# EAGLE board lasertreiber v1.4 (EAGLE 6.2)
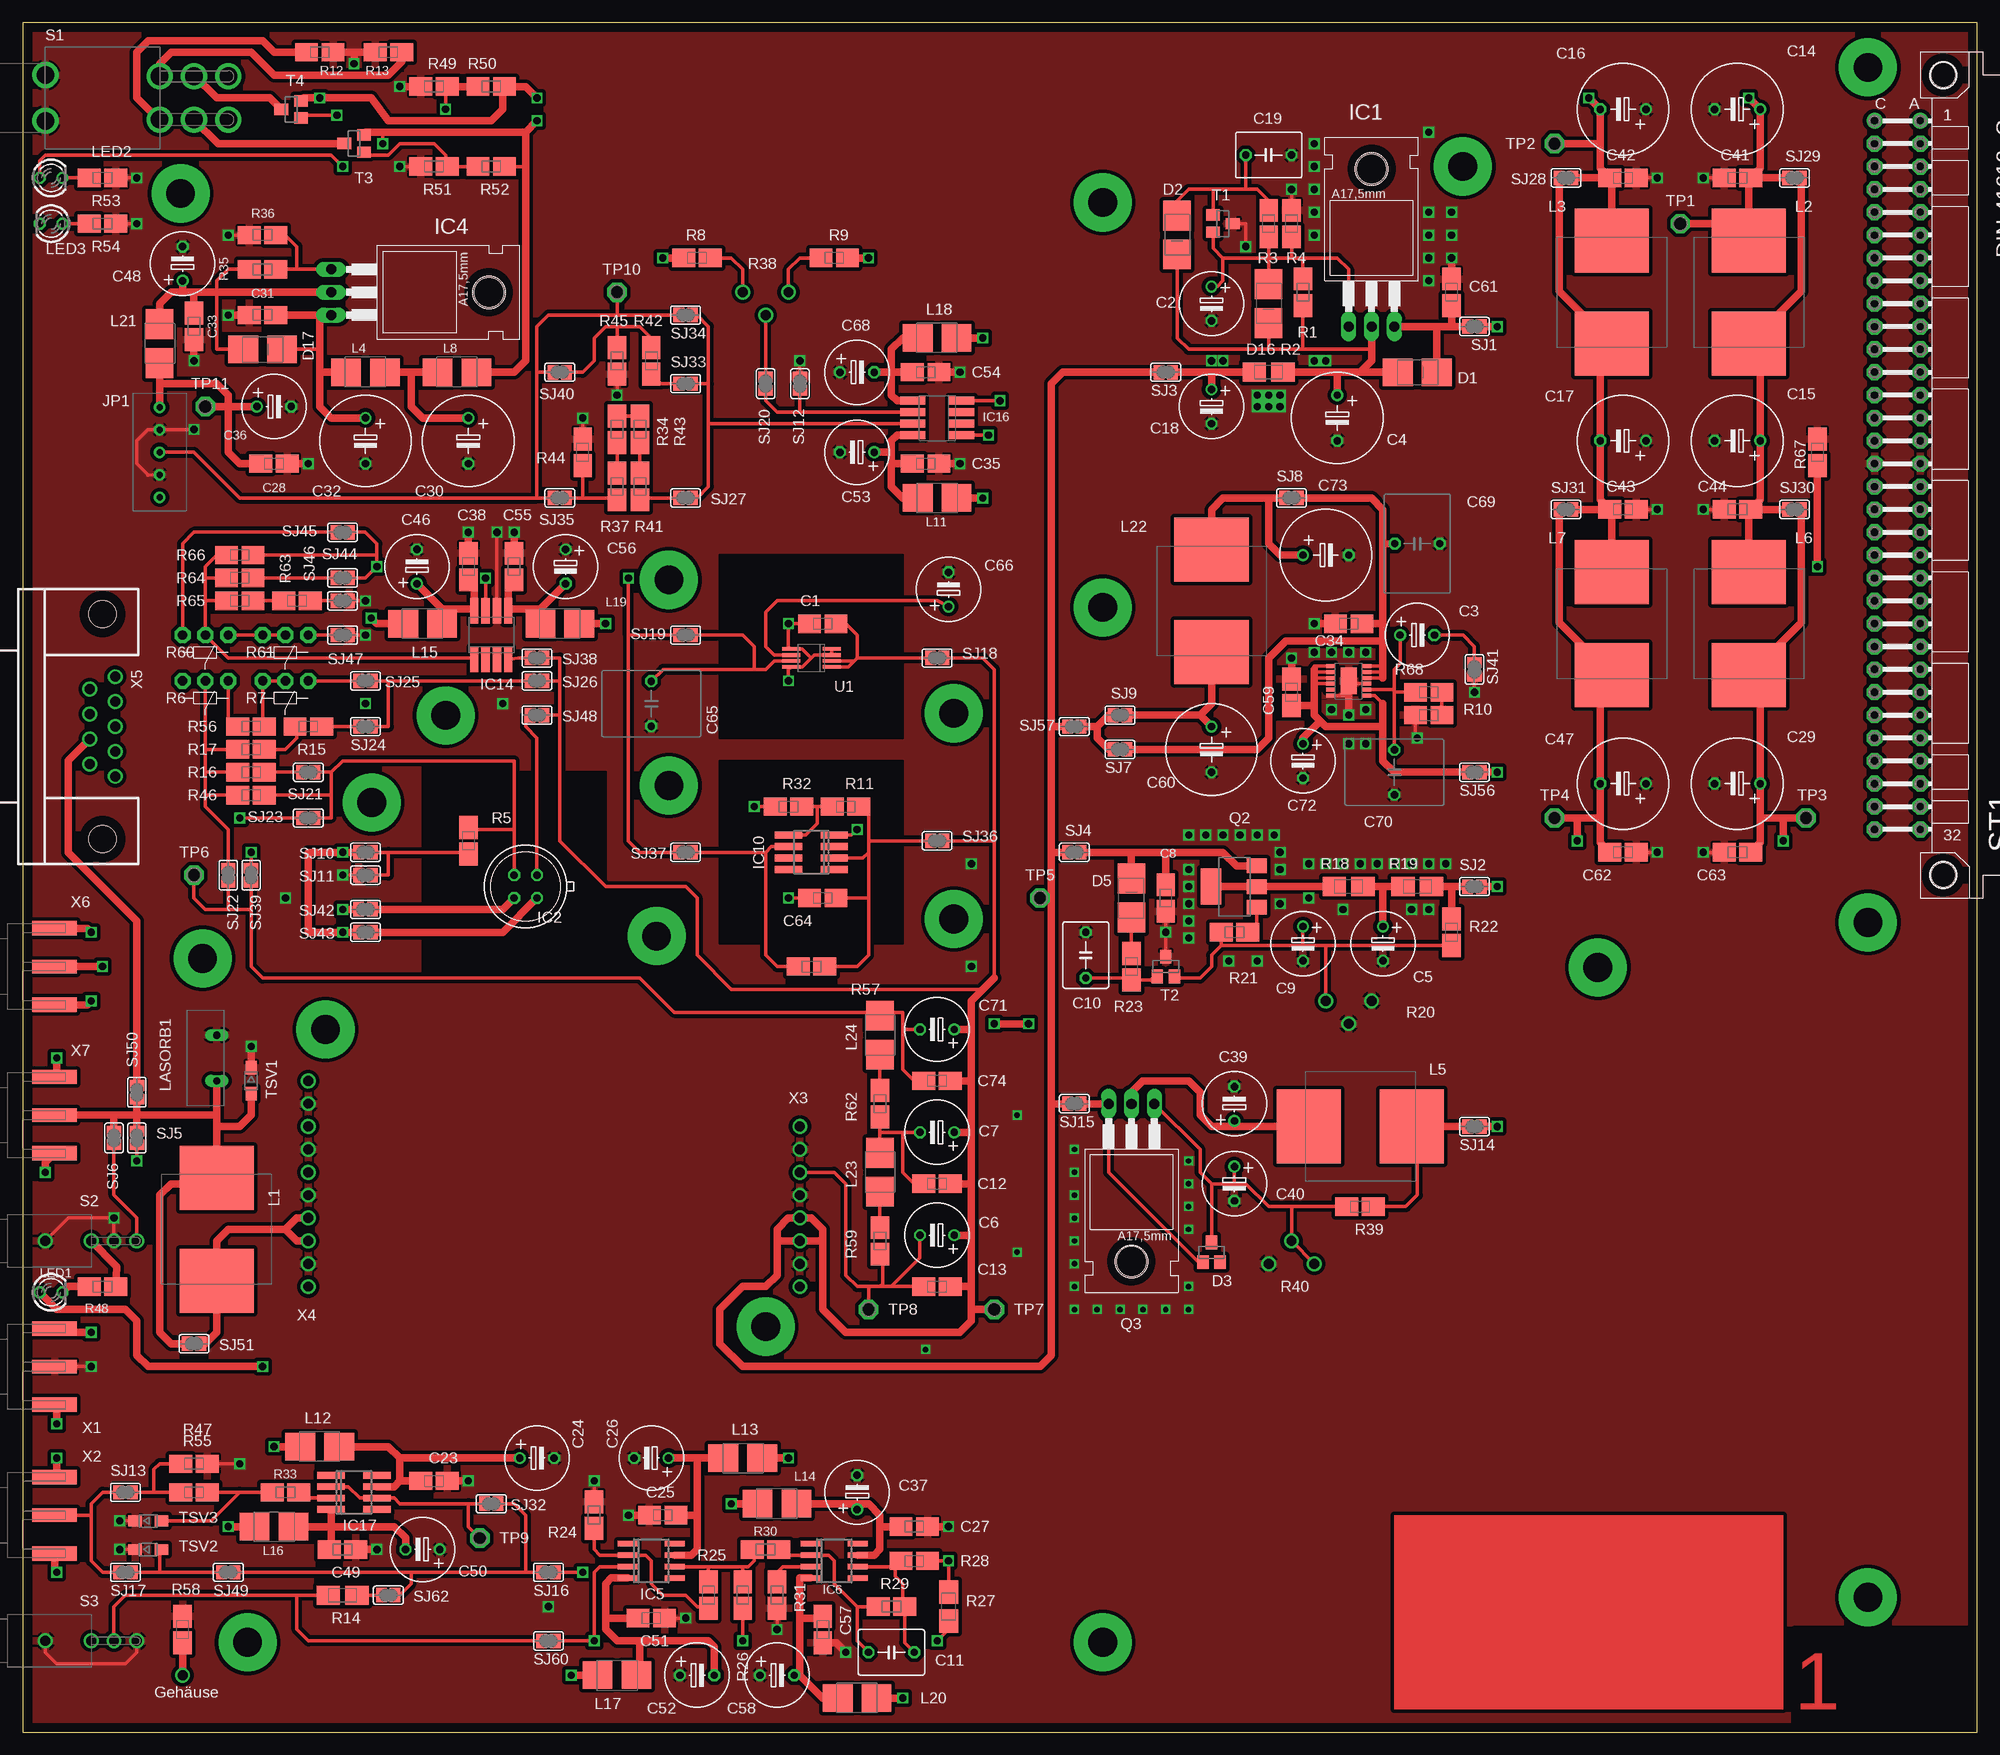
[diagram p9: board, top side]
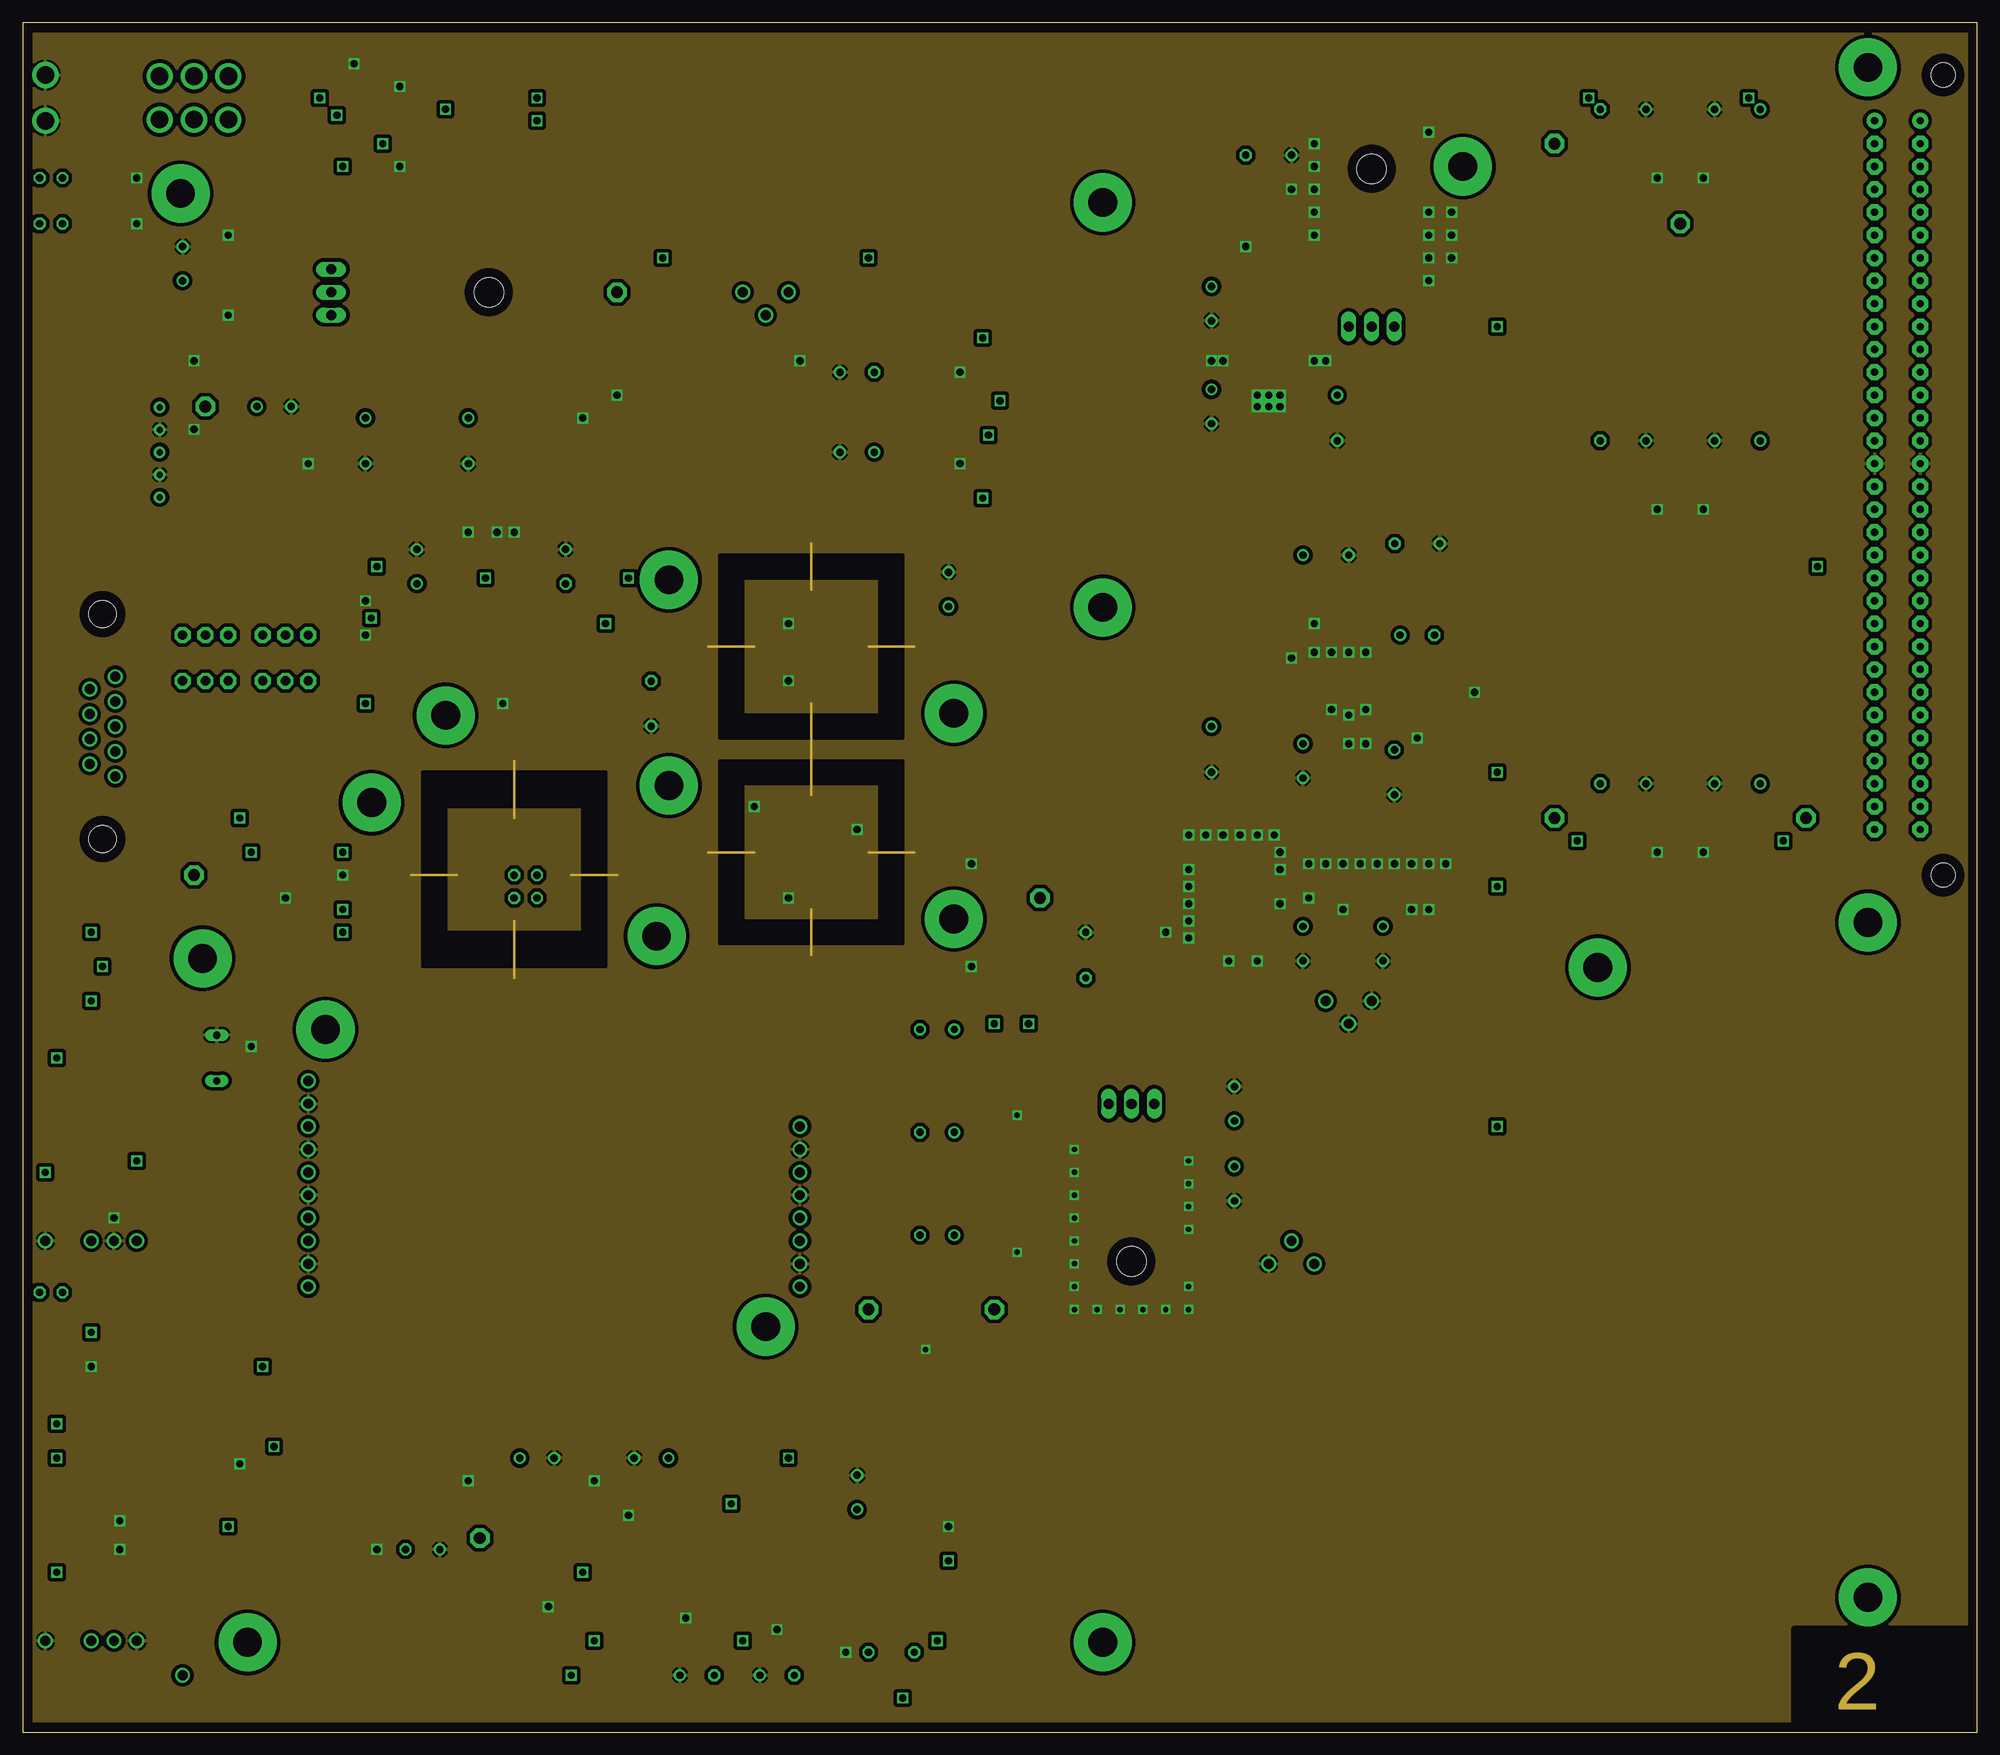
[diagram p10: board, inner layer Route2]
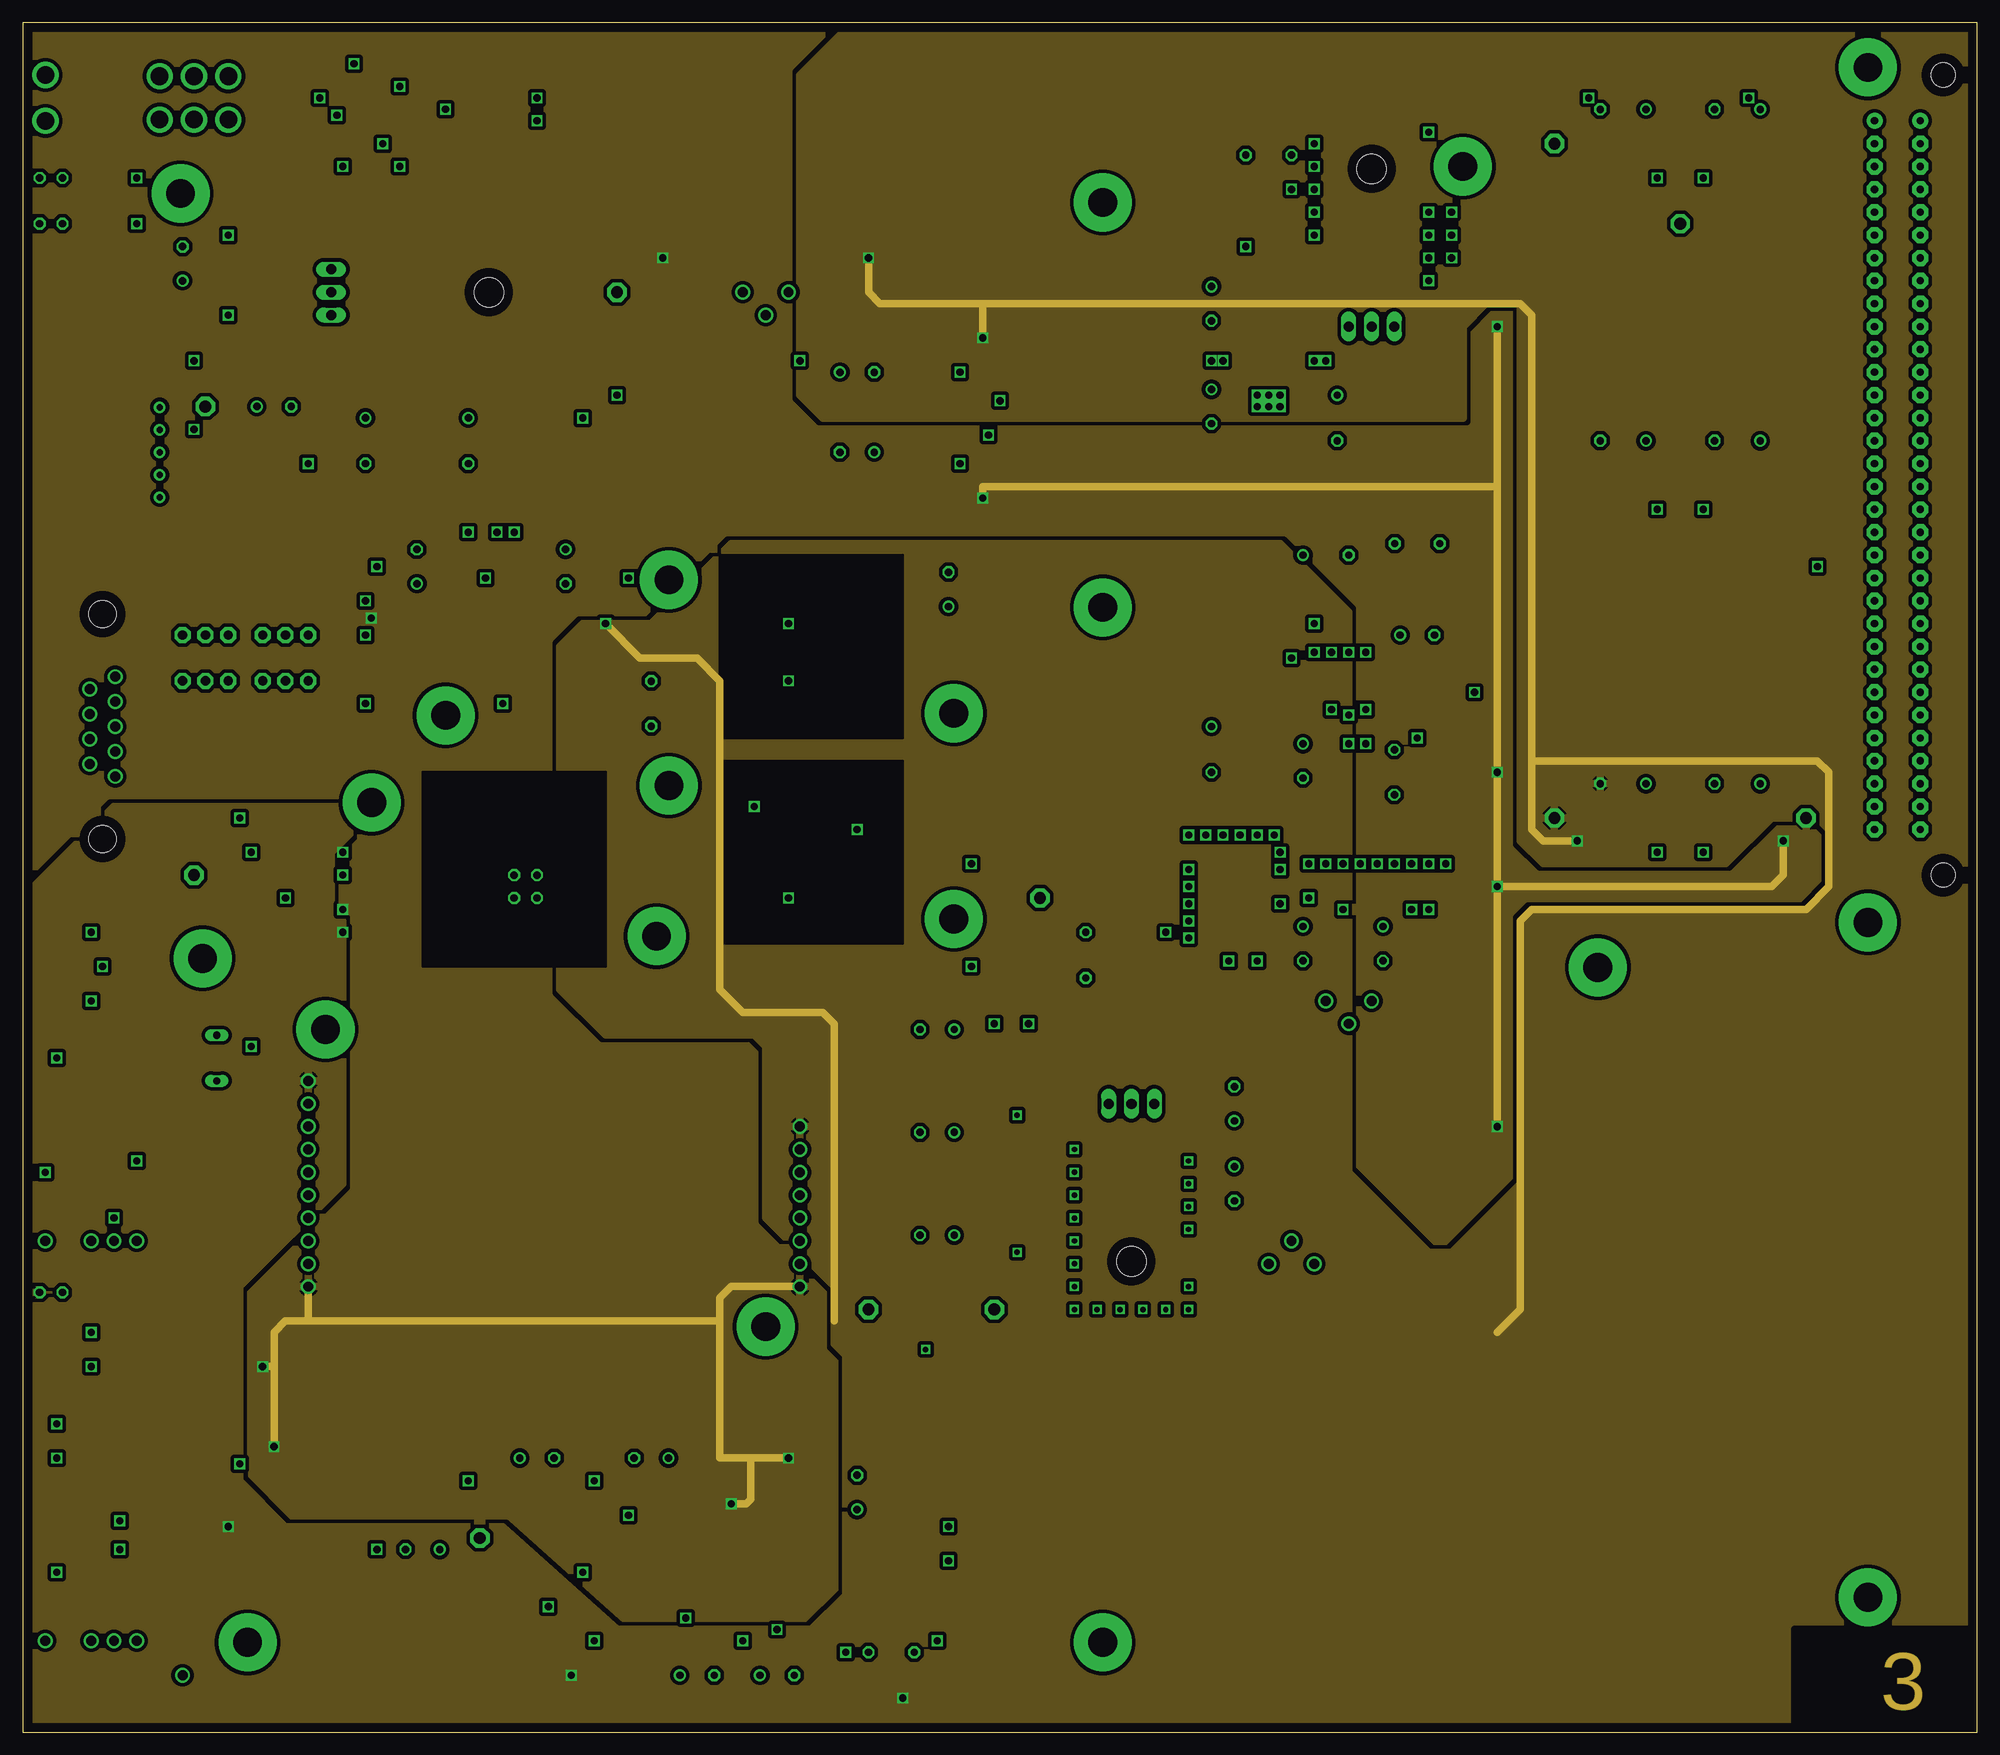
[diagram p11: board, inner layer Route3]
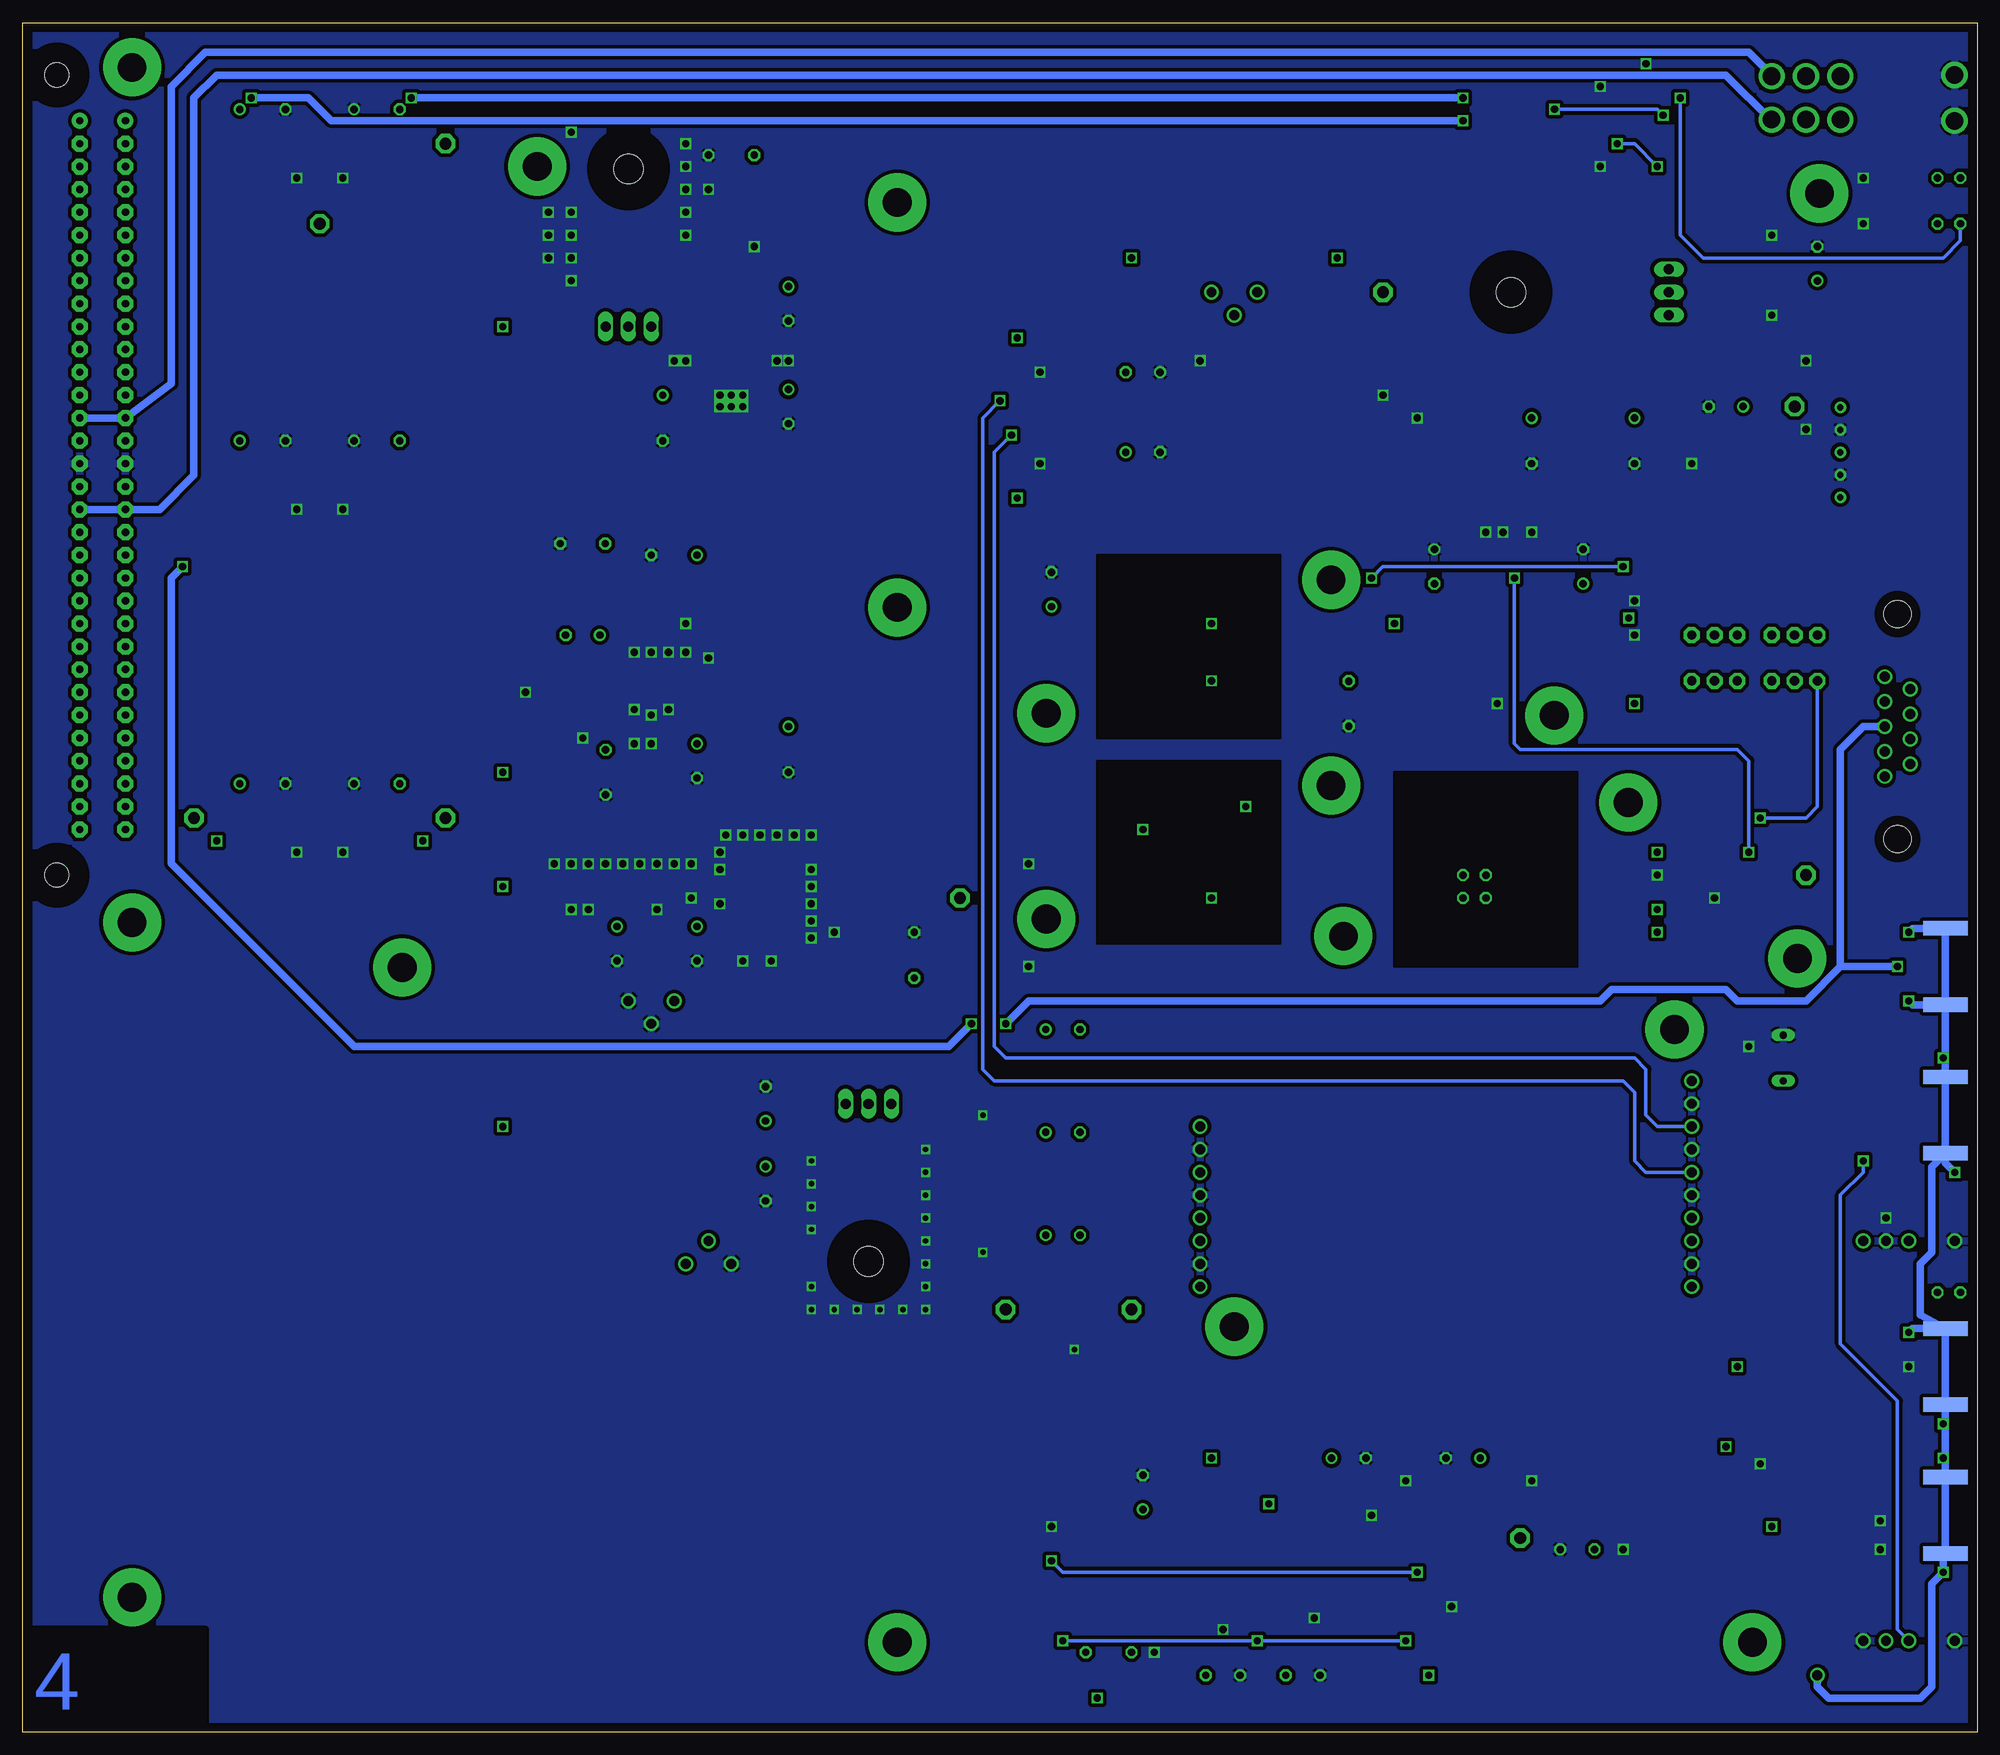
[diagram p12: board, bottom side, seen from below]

Size 217.17 x 189.99 mm. Coordinates in mm from the lower left corner, seen from the top.
Outline: 0,0 217.17,0 217.17,189.99 0,189.99 0,0
Copper layers (1+2*3+16): Top 0.018mm / dielectric 0.14mm / Route2 0.035mm / dielectric 1.2mm / Route3 0.035mm / dielectric 0.14mm / Bottom 0.018mm
Design rules: minimum track width 10mil, minimum drill 23mil, track to track 8mil, track to pad 8mil, pad to pad 8mil, via to via 8mil, smd to smd 8mil, copper to edge 40mil, drill to drill 8mil, minimum pad ring 10mil, minimum via ring 8mil, stop-mask expansion 4mil, vias tented up to drill 0mil, thermal gap 10mil

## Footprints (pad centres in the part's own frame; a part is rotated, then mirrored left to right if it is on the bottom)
LOCH-M3 = drill 3.2 pad 6.452: 1 0,0
BOX-15X15MM = drill 3.2 pad 6.452: 1 -15.824,7.417; 2 15.824,-7.417
C0805 = smd 2.54 x 2.032: 1 -1.473,0; 2 1.473,0
TT5D7 = drill 0.813: + -1.905,0 | drill 0.813 octagon: - 1.905,0
TT5D10 = drill 0.813: + -2.54,0 | drill 0.813 octagon: - 2.54,0
C050-050X075 = drill 0.813 octagon: 1 -2.54,0; 2 2.54,0
MKS2 = drill 0.813 octagon: 1 -2.5,0; 2 2.5,0
DIODE = smd 3.302 x 3.048: ANODE -2.159,0; KATHODE 2.159,0
SOT23 = smd 1.27 x 1.524: 1 -0.95,-1.1; 2 0.95,-1.1; 3 0,1.1
GEHAEUSEMASSE = drill 1.1: P$2 0,0
TO220 = drill 1.118 long: 1 -2.54,-6.35; 2 0,-6.35; 3 2.54,-6.35 | hole 3.302: 0,11.176
TO39/4 = drill 0.813 octagon: 1 -1.27,-1.27; 2 1.27,-1.27; 3 1.27,1.27; 4 -1.27,1.27
MSE = smd 0.445 x 1.016: 1 -1.626,-2; 2 -0.975,-2; 3 -0.325,-2; 4 0.325,-2; 5 0.975,-2; 6 1.626,-2; 7 1.626,2; 8 0.975,2; 9 0.325,2; 10 -0.325,2; 11 -0.975,2; 12 -1.626,2 | smd 2.9 x 1.75: 13 0,0
SO08 = smd 0.6 x 2.2: 1 -1.905,-2.6; 2 -0.635,-2.6; 3 0.635,-2.6; 4 1.905,-2.6; 5 1.905,2.6; 6 0.635,2.6; 7 -0.635,2.6; 8 -1.905,2.6
SOIC8 = smd 0.762 x 3.048: 1 -1.905,-2.54; 2 -0.635,-2.54; 3 0.635,-2.54; 4 1.905,-2.54; 5 1.905,2.54; 6 0.635,2.54; 7 -0.635,2.54; 8 -1.905,2.54
R-8 = smd 0.9 x 2.8: 1 -1.905,-2.7; 2 -0.635,-2.7; 3 0.635,-2.7; 4 1.905,-2.7; 5 1.905,2.7; 6 0.635,2.7; 7 -0.635,2.7; 8 -1.905,2.7
IL-G5 = drill 0.7 pad 1.27: P$1 0,5; P$2 0,2.5; P$3 0,0; P$4 0,-2.5; P$5 0,-5
L-GROSS = smd 7.112 x 8.23: P$1 -5.715,0; P$2 5.715,0
L-KLEIN = smd 3.302 x 3.048: 1 -2.159,0; 2 2.159,0
LASORB = drill 0.8 long: LDA 2.54,0; LDK -2.54,0
LED3MM = drill 0.813 octagon: A -1.27,0; K 1.27,0
SOT223 = smd 1.6 x 2.2: 1 -2.3,-2.5; 2 0,-2.5; 3 2.3,-2.5 | smd 4 x 2.3: 4 0,2.6
R0805 = smd 2.54 x 2.032: 1 -1.473,0; 2 1.473,0
R1206 = smd 2.6 x 2.1: 1 -1.6,0; 2 1.6,0
PT-10 = drill 1.016 pad 1.778 octagon: 1 -2.54,1.27; 2 2.54,1.27; 3 0,1.27
64Y-POTI = drill 1.1: 1 2.54,-1.27; 2 0,1.27; 3 -2.54,-1.27
1MD1T2B4M7QE = drill 1.95: 1 -2.413,0; 2 -2.413,3.81; 3 -2.413,7.62; 4 2.413,0; 5 2.413,3.81; 6 2.413,7.62; 7 -2.54,-12.7; 8 2.54,-12.7
2AS1T2A1M7RE = drill 1.1: 1 0,0; 2 0,2.54; 3 0,5.08; 4 0,-5.08
SJ = smd 1.168 x 1.6: 1 -0.762,0; 2 0.762,0
A.KO-09_MAC64L = drill 0.8 pad 1.778: A1 -1.27,39.37; C1 -6.35,39.37 | drill 0.8 pad 1.778 octagon: A2 -1.27,36.83; A3 -1.27,34.29; A4 -1.27,31.75; A5 -1.27,29.21; A6 -1.27,26.67; A7 -1.27,24.13; A8 -1.27,21.59; A9 -1.27,19.05; A10 -1.27,16.51; A11 -1.27,13.97; A12 -1.27,11.43; A13 -1.27,8.89; A14 -1.27,6.35; A15 -1.27,3.81; A16 -1.27,1.27; A17 -1.27,-1.27; A18 -1.27,-3.81; A19 -1.27,-6.35; A20 -1.27,-8.89; A21 -1.27,-11.43; A22 -1.27,-13.97; A23 -1.27,-16.51; A24 -1.27,-19.05; A25 -1.27,-21.59; A26 -1.27,-24.13; A27 -1.27,-26.67; A28 -1.27,-29.21; A29 -1.27,-31.75; A30 -1.27,-34.29; A31 -1.27,-36.83; A32 -1.27,-39.37; C2 -6.35,36.83; C3 -6.35,34.29; C4 -6.35,31.75; C5 -6.35,29.21; C6 -6.35,26.67; C7 -6.35,24.13; C8 -6.35,21.59; C9 -6.35,19.05; C10 -6.35,16.51; C11 -6.35,13.97; C12 -6.35,11.43; C13 -6.35,8.89; C14 -6.35,6.35; C15 -6.35,3.81; C16 -6.35,1.27; C17 -6.35,-1.27; C18 -6.35,-3.81; C19 -6.35,-6.35; C20 -6.35,-8.89; C21 -6.35,-11.43; C22 -6.35,-13.97; C23 -6.35,-16.51; C24 -6.35,-19.05; C25 -6.35,-21.59; C26 -6.35,-24.13; C27 -6.35,-26.67; C28 -6.35,-29.21; C29 -6.35,-31.75; C30 -6.35,-34.29; C31 -6.35,-36.83; C32 -6.35,-39.37 | hole 2.7: 1.27,44.45; 1.27,-44.45
P1-13 = drill 1.321 pad 2.159 octagon: TP 0,0
SOD323-W = smd 1.5 x 1.2: A 1.45,0; C -1.45,0
MS8 = smd 0.4 x 2: 1 -1,-2.25; 2 -0.325,-2.25; 3 0.325,-2.25; 4 1,-2.25; 5 1,2.25; 6 0.325,2.25; 7 -0.325,2.25; 8 -1,2.25
SMA20_HRZ = smd 1.6 x 4.902 bottom: GND@1 -4.242,3.556; GND@4 4.242,3.556 | smd 1.6 x 4.902: GND@2 -4.242,3.556; GND@3 4.242,3.556 | smd 1.499 x 4.902: SIGNAL 0,3.556
PINHEADER-8 = drill 1.1: 1 -8.89,0; 2 -6.35,0; 3 -3.81,0; 4 -1.27,0; 5 1.27,0; 6 3.81,0; 7 6.35,0; 8 8.89,0
PINHEADER-10 = drill 1.1: 1 -11.43,0; 2 -8.89,0; 3 -6.35,0; 4 -3.81,0; 5 -1.27,0; 6 1.27,0; 7 3.81,0; 8 6.35,0; 9 8.89,0; 10 11.43,0
H3M09RA = drill 1.092: 1 -5.537,1.422; 2 -2.769,1.422; 3 0,1.422; 4 2.769,1.422; 5 5.537,1.422; 6 -4.153,-1.422; 7 -1.384,-1.422; 8 1.384,-1.422; 9 4.153,-1.422 | hole 3.048: -12.497,0; 12.497,0

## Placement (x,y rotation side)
BOLZEN1  BOLZEN-M3  [LOCH-M3]  17.56,171 0 top
BOLZEN2  BOLZEN-M3  [LOCH-M3]  25,10 0 top
BOLZEN3  BOLZEN-M3  [LOCH-M3]  47,113 0 top
BOLZEN4  BOLZEN-M3  [LOCH-M3]  120,10 0 top
BOLZEN5  BOLZEN-M3  [LOCH-M3]  120,125 0 top
BOLZEN6  BOLZEN-M3  [LOCH-M3]  205,15 0 top
BOLZEN7  BOLZEN-M3  [LOCH-M3]  120,170 0 top
BOLZEN8  BOLZEN-M3  [LOCH-M3]  205,90 0 top
BOLZEN9  BOLZEN-M3  [LOCH-M3]  160,174 270 top
BOLZEN10  BOLZEN-M3  [LOCH-M3]  20,86 0 top
BOLZEN11  BOLZEN-M3  [LOCH-M3]  175,85 0 top
BOLZEN12  BOLZEN-M3  [LOCH-M3]  205,185 0 top
BOLZEN13  BOLZEN-M3  [LOCH-M3]  82.55,45.09 90 top
BOLZEN14  BOLZEN-M3  [LOCH-M3]  33.66,78.11 0 top
BOX1  BOX15X15MM  [BOX-15X15MM]  54.61,95.89 0 top
BOX2  BOX15X15MM  [BOX-15X15MM]  87.63,120.65 0 top
BOX3  BOX15X15MM  [BOX-15X15MM]  87.63,97.79 0 top
C1  100n  [C0805]  88.9,123.19 180 top
C2  100u  [TT5D7]  132.08,158.75 270 top
C3  100u  [TT5D7]  154.94,121.92 0 top
C4  1000u  [TT5D10]  146.05,146.05 270 top
C5  100u  [TT5D7]  151.13,87.63 270 top
C6  100u  [TT5D7]  101.6,55.24 180 top
C7  100u  [TT5D7]  101.6,66.67 180 top
C8  100n  [C0805]  127,92.71 90 top
C9  100u  [TT5D7]  142.24,87.63 270 top
C10  1u  [C050-050X075]  118.11,86.36 270 top
C11  1u  [C050-050X075]  96.52,8.89 0 top
C12  100n  [C0805]  101.6,60.96 0 top
C13  100n  [C0805]  101.6,49.53 0 top
C14  1000u  [TT5D10]  190.5,180.34 180 top
C15  1000u  [TT5D10]  190.5,143.51 180 top
C16  1000u  [TT5D10]  177.8,180.34 180 top
C17  1000u  [TT5D10]  177.8,143.51 180 top
C18  100u  [TT5D7]  132.08,147.32 270 top
C19  1u  [C050-050X075]  138.43,175.26 180 top
C23  100n  [C0805]  45.72,27.94 0 top
C24  100u  [TT5D7]  57.15,30.48 0 top
C25  100n  [C0805]  71.12,24.13 180 top
C26  100u  [TT5D7]  69.85,30.48 180 top
C27  100n  [C0805]  99.06,22.86 0 top
C28  100n  [C0805]  27.94,140.97 0 top
C29  1000u  [TT5D10]  190.5,105.41 180 top
C30  1000u  [TT5D10]  49.53,143.51 270 top
C31  100n  [C0805]  26.67,157.48 180 top
C32  1000u  [TT5D10]  38.1,143.51 270 top
C33  100n  [C0805]  19.05,156.21 270 top
C34  100n  [C0805]  147.32,123.19 0 top
C35  100n  [C0805]  100.33,140.97 0 top
C36  100u  [TT5D7]  27.94,147.32 0 top
C37  100u  [TT5D7]  92.71,26.67 90 top
C38  100n  [C0805]  49.53,129.54 90 top
C39  100u  [TT5D7]  134.62,69.85 90 top
C40  100u  [TT5D7]  134.62,60.96 270 top
C41  100n  [C0805]  190.5,172.72 180 top
C42  100n  [C0805]  177.8,172.72 180 top
C43  100n  [C0805]  177.8,135.89 180 top
C44  100n  [C0805]  190.5,135.89 180 top
C46  100u  [TT5D7]  43.81,129.54 90 top
C47  1000u  [TT5D10]  177.8,105.41 180 top
C48  100u  [TT5D7]  17.78,163.19 90 top
C49  100n  [C0805]  35.56,20.32 0 top
C50  100u  [TT5D7]  44.45,20.32 180 top
C51  100n  [C0805]  69.85,12.7 0 top
C52  100u  [TT5D7]  74.93,6.35 0 top
C53  100u  [TT5D7]  92.71,142.24 180 top
C54  100n  [C0805]  100.33,151.13 0 top
C55  100n  [C0805]  54.61,129.54 90 top
C56  100u  [TT5D7]  60.33,129.54 270 top
C57  100n  [C0805]  88.9,11.43 270 top
C58  100u  [TT5D7]  83.82,6.35 0 top
C59  100n  [C0805]  140.97,115.57 270 top
C60  1000u  [TT5D10]  132.08,109.22 270 top
C61  100n  [C0805]  158.75,160.02 270 top
C62  100n  [C0805]  177.8,97.79 180 top
C63  100n  [C0805]  190.5,97.79 180 top
C64  100n  [C0805]  88.9,92.71 180 top
C65  10u  [MKS2]  69.85,114.3 270 top
C66  100u  [TT5D7]  102.87,127 90 top
C68  100u  [TT5D7]  92.71,151.13 0 top
C69  10u  [MKS2]  154.94,132.08 180 top
C70  10u  [MKS2]  152.4,106.68 90 top
C71  100u  [TT5D7]  101.6,78.11 180 top
C72  100u  [TT5D7]  142.24,107.95 270 top
C73  1000u  [TT5D10]  144.78,130.81 0 top
C74  100n  [C0805]  101.6,72.39 0 top
D1  DIODEM6  [DIODE]  154.94,151.13 0 top
D2  DIODEM6  [DIODE]  128.27,166.37 270 top
D3  BZX84-A12  [SOT23]  132.08,53.34 0 top
D5  DIODEM6  [DIODE]  123.19,92.71 90 top
D16  DIODEM6  [DIODE]  138.43,158.75 270 top
D17  DIODEM6  [DIODE]  26.67,153.67 0 top
GEHAEUSE1  GEHAEUSEMASSE  [GEHAEUSEMASSE]  17.78,6.35 0 top
IC1  LM317KCS  [TO220]  149.86,162.56 0 top
IC2  LM399H  [TO39/4]  55.88,93.98 180 top
IC3  LT3045  [MSE]  147.32,116.84 270 top
IC4  LM317KCS  [TO220]  40.64,160.02 270 top
IC5  OP27D  [SO08]  69.85,19.05 270 top
IC6  OP27D  [SO08]  90.17,19.05 270 top
IC10  LT1236S-10  [SOIC8]  87.63,97.79 90 top
IC14  AD8429  [R-8]  52.07,121.92 0 top
IC16  AD8429  [R-8]  101.6,146.05 90 top
IC17  LT1028  [SOIC8]  36.83,26.67 270 top
JP1  IL-G5  [IL-G5]  15.24,142.24 180 top
L1  100u  [L-GROSS]  21.59,55.88 90 top
L2  100u  [L-GROSS]  191.77,160.02 270 top
L3  100u  [L-GROSS]  176.53,160.02 270 top
L4  100u  [L-KLEIN]  38.1,151.13 180 top
L5  100u  [L-GROSS]  148.59,67.31 180 top
L6  100u  [L-GROSS]  191.77,123.19 270 top
L7  100u  [L-GROSS]  176.53,123.19 270 top
L8  100u  [L-KLEIN]  48.26,151.13 180 top
L11  100u  [L-KLEIN]  101.6,137.16 0 top
L12  100u  [L-KLEIN]  33.02,31.75 180 top
L13  100u  [L-KLEIN]  80.01,30.48 0 top
L14  100u  [L-KLEIN]  83.82,25.4 180 top
L15  100u  [L-KLEIN]  44.45,123.19 180 top
L16  100u  [L-KLEIN]  27.94,22.86 0 top
L17  100u  [L-KLEIN]  66.04,6.35 0 top
L18  100u  [L-KLEIN]  101.6,154.94 180 top
L19  100u  [L-KLEIN]  59.69,123.19 180 top
L20  100u  [L-KLEIN]  92.71,3.81 180 top
L21  100u  [L-KLEIN]  15.24,154.31 270 top
L22  100u  [L-GROSS]  132.08,125.73 270 top
L23  100u  [L-KLEIN]  95.25,62.23 270 top
L24  100u  [L-KLEIN]  95.25,77.47 270 top
LASORB1  LASORB  [LASORB]  21.59,74.93 270 top
LED1  GRUEN  [LED3MM]  3.17,48.9 0 top
LED2  GRUEN  [LED3MM]  3.17,172.72 0 top
LED3  GRUEN  [LED3MM]  3.17,167.64 180 top
Q2  BCP56  [SOT223]  134.62,93.98 90 top
Q3  IRF512  [TO220]  123.19,63.5 180 top
R1  330R  [R0805]  142.24,160.02 270 top
R2  4R7  [R1206]  138.43,151.13 0 top
R3  51k  [R0805]  138.43,167.64 90 top
R4  3k3  [R0805]  140.97,167.64 270 top
R5  7.5k  [R0805]  49.53,99.06 90 top
R6  10k  [PT-10]  20.32,115.57 0 top
R7  100k  [PT-10]  29.21,115.57 0 top
R8  10k  [R0805]  74.93,163.83 180 top
R9  10k  [R0805]  90.17,163.83 180 top
R10  20k  [R0805]  156.21,113.03 0 top
R11  4k7  [R0805]  91.44,102.87 180 top
R12  10R  [R0805]  33.02,186.69 0 top
R13  10R  [R0805]  40.64,186.69 180 top
R14  1k  [R1206]  35.56,15.24 0 top
R15  [R0805]  31.75,111.76 0 top
R16  [R0805]  25.4,106.68 180 top
R17  [R0805]  25.4,109.22 0 top
R18  4R7  [R1206]  147.32,93.98 0 top
R19  4R7  [R1206]  154.94,93.98 0 top
R20  10k  [64Y-POTI]  147.32,80.01 180 top
R21  10R  [R0805]  134.62,88.9 180 top
R22  10k  [R0805]  158.75,88.9 90 top
R23  51k  [R0805]  123.19,85.09 270 top
R24  1k  [R0805]  63.5,24.13 90 top
R25  1k  [R0805]  76.2,15.24 270 top
R26  1k  [R0805]  80.01,15.24 270 top
R27  1k  [R1206]  102.87,13.97 90 top
R28  2k  [R0805]  99.06,19.05 180 top
R29  1k  [R0805]  96.52,13.97 180 top
R30  1k  [R0805]  82.55,20.32 180 top
R31  1k  [R0805]  83.82,15.24 270 top
R32  4k7  [R0805]  85.09,102.87 180 top
R33  250R  [R0805]  29.21,26.67 0 top
R34  10k  [R0805]  66.04,144.78 90 top
R35  330R  [R0805]  26.67,162.56 180 top
R36  1k  [R0805]  26.67,166.37 0 top
R37  10k  [R0805]  66.04,138.43 90 top
R38  1k  [64Y-POTI]  82.55,158.75 180 top
R39  1k  [R0805]  148.59,58.42 0 top
R40  100k  [64Y-POTI]  140.97,53.34 0 top
R41  10k  [R0805]  68.58,138.43 270 top
R42  10k  [R0805]  69.85,152.4 270 top
R43  10k  [R0805]  68.58,144.78 270 top
R44  10k  [R0805]  62.23,142.24 270 top
R45  10k  [R0805]  66.04,152.4 90 top
R46  1M  [R0805]  25.4,104.14 180 top
R47  49R9  [R0805]  19.05,29.84 180 top
R48  10k  [R0805]  8.89,49.53 0 top
R49  100k  [R0805]  45.72,182.88 180 top
R50  100k  [R0805]  52.07,182.88 180 top
R51  100k  [R0805]  45.72,173.99 0 top
R52  100k  [R0805]  52.07,173.99 0 top
R53  10k  [R0805]  8.89,172.72 0 top
R54  10k  [R0805]  8.89,167.64 0 top
R55  250R  [R0805]  19.05,26.67 0 top
R56  [R0805]  25.4,111.76 0 top
R57  1M  [R0805]  87.63,85.09 180 top
R58  0R  [R0805]  17.78,11.43 90 top
R59  1k  [R0805]  95.25,54.61 270 top
R60  10k  [PT-10]  20.32,120.65 0 top
R61  100k  [PT-10]  29.21,120.65 0 top
R62  1k  [R0805]  95.25,69.85 270 top
R63  [R0805]  30.48,125.73 0 top
R64  [R0805]  24.13,128.27 180 top
R65  [R0805]  24.13,125.73 0 top
R66  1M  [R0805]  24.13,130.81 180 top
R67  0R  [R0805]  199.39,142.24 90 top
R68  100k  [R0805]  156.21,115.57 180 top
S1  1MD1T2B4M7QE  [1MD1T2B4M7QE]  15.24,181.61 270 top
S2  2AS1T2A1M7RE  [2AS1T2A1M7RE]  7.62,54.61 270 top
S3  2AS1T2A1M7RE  [2AS1T2A1M7RE]  7.62,10.16 270 top
SJ1  [SJ]  161.29,156.21 180 top
SJ2  [SJ]  161.29,93.98 180 top
SJ3  [SJ]  127,151.13 180 top
SJ4  [SJ]  116.84,97.79 180 top
SJ5  [SJ]  12.7,66.04 90 top
SJ6  [SJ]  10.16,66.04 270 top
SJ7  [SJ]  121.92,109.22 180 top
SJ8  [SJ]  140.97,137.16 180 top
SJ9  [SJ]  121.92,113.03 180 top
SJ10  [SJ]  38.1,97.79 180 top
SJ11  [SJ]  38.1,95.25 180 top
SJ12  [SJ]  86.36,149.86 90 top
SJ13  [SJ]  11.43,26.67 0 top
SJ14  [SJ]  161.29,67.31 180 top
SJ15  [SJ]  116.84,69.85 180 top
SJ16  [SJ]  58.42,17.78 0 top
SJ17  [SJ]  11.43,17.78 0 top
SJ18  [SJ]  101.6,119.38 0 top
SJ19  [SJ]  73.66,121.92 180 top
SJ20  [SJ]  82.55,149.86 90 top
SJ21  [SJ]  31.75,106.68 180 top
SJ22  [SJ]  22.86,95.25 270 top
SJ23  [SJ]  31.75,101.6 180 top
SJ24  [SJ]  38.1,111.76 0 top
SJ25  [SJ]  38.1,116.84 0 top
SJ26  [SJ]  57.15,116.84 0 top
SJ27  [SJ]  73.66,137.16 180 top
SJ28  [SJ]  171.45,172.72 180 top
SJ29  [SJ]  196.85,172.72 0 top
SJ30  [SJ]  196.85,135.89 0 top
SJ31  [SJ]  171.45,135.89 180 top
SJ32  [SJ]  52.07,25.4 0 top
SJ33  [SJ]  73.66,149.86 180 top
SJ34  [SJ]  73.66,157.48 180 top
SJ35  [SJ]  59.69,137.16 180 top
SJ36  [SJ]  101.6,99.06 0 top
SJ37  [SJ]  73.66,97.79 180 top
SJ38  [SJ]  57.15,119.38 180 top
SJ39  [SJ]  25.4,95.25 270 top
SJ40  [SJ]  59.69,151.13 180 top
SJ41  [SJ]  161.29,118.11 90 top
SJ42  [SJ]  38.1,91.44 180 top
SJ43  [SJ]  38.1,88.9 0 top
SJ44  [SJ]  35.56,128.27 180 top
SJ45  [SJ]  35.56,133.35 180 top
SJ46  [SJ]  35.56,125.73 0 top
SJ47  [SJ]  35.56,121.92 0 top
SJ48  [SJ]  57.15,113.03 0 top
SJ49  [SJ]  22.86,17.78 0 top
SJ50  [SJ]  12.7,71.12 90 top
SJ51  [SJ]  19.05,43.18 0 top
SJ56  [SJ]  161.29,106.68 180 top
SJ57  [SJ]  116.84,111.76 180 top
SJ60  [SJ]  58.42,10.16 180 top
SJ62  [SJ]  40.64,15.24 180 top
ST1  [A.KO-09_MAC64L]  212.09,139.7 0 top
T1  BC857C  [SOT23]  133.35,167.64 270 top
T2  BC857C  [SOT23]  127,85.09 0 top
T3  IRLML9301  [SOT23]  36.83,176.53 90 top
T4  IRLML0060  [SOT23]  29.84,180.34 90 top
TP1  PTR1PAD1-13  [P1-13]  184.15,167.64 0 top
TP2  PTR1PAD1-13  [P1-13]  170.18,176.53 0 top
TP3  PTR1PAD1-13  [P1-13]  198.12,101.6 0 top
TP4  PTR1PAD1-13  [P1-13]  170.18,101.6 0 top
TP5  PTR1PAD1-13  [P1-13]  113.03,92.71 0 top
TP6  PTR1PAD1-13  [P1-13]  19.05,95.25 270 top
TP7  PTR1PAD1-13  [P1-13]  107.95,46.99 0 top
TP8  PTR1PAD1-13  [P1-13]  93.98,46.99 0 top
TP9  PTR1PAD1-13  [P1-13]  50.8,21.59 0 top
TP10  PTR1PAD1-13  [P1-13]  66.04,160.02 0 top
TP11  PTR1PAD1-13  [P1-13]  20.32,147.32 0 top
TSV1  CDSOD323-T03SC  [SOD323-W]  25.4,72.39 270 top
TSV2  CDSOD323-T12C-DSL  [SOD323-W]  13.97,20.32 0 top
TSV3  CDSOD323-T12C-DSL  [SOD323-W]  13.97,23.5 0 top
U1  LTC6655LNBHMS8-5  [MS8]  87.63,119.38 90 top
X1  SMAHRZ  [SMA20_HRZ]  0,40.64 270 top
X2  SMAHRZ  [SMA20_HRZ]  0,24.13 270 top
X3  PINHEADER-8  [PINHEADER-8]  86.36,58.42 90 top
X4  PINHEADER-10  [PINHEADER-10]  31.75,60.96 270 top
X5  D-SUB9-H3M09RA  [H3M09RA]  8.89,111.76 270 top
X6  SMAHRZ  [SMA20_HRZ]  0,85.09 270 top
X7  SMAHRZ  [SMA20_HRZ]  0,68.58 270 top

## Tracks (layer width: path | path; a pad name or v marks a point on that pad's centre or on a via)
+15V  (via drill 0.8)
  Top 0.813: SJ30.2 197.61,123.32 L6.P$2 193.04,116.2 C29.+ 193.04,101.6 | 193.04,101.6 193.04,98.86 C63.1 | R8.2 v71.12,163.83 | SJ42.2 v35.56,91.44 | 193.04,101.6 195.58,101.6 | 195.58,101.6 TP3.TP | SJ1.1 v163.83,156.21 | v163.83,106.68 SJ56.1 | v163.83,93.98 SJ2.1 | v163.83,67.31 SJ14.1 | v195.58,99.06 195.58,101.6 | L12.2 v27.94,31.75 | v85.09,30.48 L13.2 | v78.74,25.4 L14.2 | L11.2 v106.68,137.16 | LED1.A 3.81,46.99 11.43,46.99 12.7,45.72 12.7,41.91 13.97,40.64 v26.67,40.64 | L15.2 39.37,123.19 v38.73,123.83
  Route3 0.813: v163.83,156.21 163.83,138.43 | 163.83,138.43 v163.83,106.68 v163.83,93.98 | v163.83,93.98 v163.83,67.31 | v163.83,93.98 194.31,93.98 195.58,95.25 v195.58,99.06 | 80.9,30.48 v85.09,30.48 | 80.9,30.48 80.9,25.91 80.39,25.4 v78.74,25.4 | 31.75,45.72 29.21,45.72 27.94,44.45 27.94,40.64 | 31.75,45.72 77.47,45.72 | 163.83,138.43 106.68,138.43 v106.68,137.16 | v27.94,31.75 27.94,40.64 | 77.47,45.72 77.47,30.48 80.9,30.48 | v26.67,40.64 27.94,40.64 | X4.10 31.75,45.72 | X3.1 78.74,49.53 77.47,48.26 77.47,45.72
  pour Route3 (isolate 0.406, rank 3): 215.9,1.27 1.27,1.27 1.27,189.23 215.9,189.23
-15V  (via drill 0.8)
  Top 0.813: SJ31.2 170.69,123.32 L7.P$2 175.26,116.2 C47.- 175.26,101.6 | C62.2 175.26,98.86 175.26,101.6 | TP4.TP 172.72,101.6 | 172.72,101.6 175.26,101.6 | v172.72,99.06 172.72,101.6 | v93.98,163.83 R9.1 | v35.56,97.79 SJ10.2 31.75,97.79 31.75,88.9 v35.56,88.9 SJ43.1 | L16.1 v22.86,22.86 | v97.79,3.81 L20.1 | L17.1 v60.96,6.35 | L19.1 61.85,122.81 | 61.85,122.3 61.85,122.81 | 61.85,122.81 62.23,123.19 v64.77,123.19 | L18.1 v106.68,154.94
  Route3 0.813: 106.68,158.75 95.25,158.75 93.98,160.02 v93.98,163.83 | 106.68,158.75 166.37,158.75 167.64,157.48 167.64,107.95 | v172.72,99.06 168.91,99.06 167.64,100.33 167.64,107.95 | 90.17,45.72 90.17,78.74 88.9,80.01 80.01,80.01 77.47,82.55 77.47,116.84 74.93,119.38 68.58,119.38 v64.77,123.19 | 163.83,44.45 166.37,46.99 166.37,90.17 167.64,91.44 198.12,91.44 200.66,93.98 200.66,106.68 199.39,107.95 167.64,107.95 | v106.68,154.94 106.68,158.75
  pour Route3 (isolate 0.406, rank 2): 86.36,184.15 86.36,148.59 88.9,146.05 160.02,146.05 160.02,156.21 162.56,158.75 166.37,158.75 166.37,99.06 168.91,96.52 189.23,96.52 194.31,101.6 199.39,101.6 200.66,100.33 200.66,93.98 198.12,91.44 167.64,91.44 166.37,90.17 166.37,60.96 158.75,53.34 156.21,53.34 147.32,62.23 147.32,124.46 139.7,132.08 78.74,132.08 69.85,123.19 62.23,123.19 59.69,120.65 59.69,82.55 64.77,77.47 81.28,77.47 82.55,76.2 82.55,57.15 90.17,49.53 90.17,43.18 91.44,41.91 91.44,15.24 87.63,11.43 66.04,11.43 53.34,22.86 29.21,22.86 24.13,27.94 24.13,49.53 35.56,60.96 35.56,90.17 34.29,91.44 34.29,97.79 36.83,100.33 36.83,101.6 35.56,102.87 10.16,102.87 1.27,93.98 1.27,1.27 215.9,1.27 215.9,189.23 91.44,189.23
DISP_IN+
  Top 0.406: SJ34.2 66.04,157.48 | 66.04,157.48 58.42,157.48 57.15,156.21 57.15,151.13 | 57.15,151.13 SJ40.2 | SJ35.2 57.15,137.16 | 57.15,137.16 57.15,151.13 | JP1.P$3 19.05,142.24 24.13,137.16 57.15,137.16 | TP10.TP 66.04,157.48
DISP_V+
  Top 0.406: D17.ANODE 21.59,153.67 21.59,160.02 21.59,161.29 22.86,162.56 R35.2
  Top 0.813: IC4.2 21.59,160.02 19.05,160.02 | 19.05,160.02 17.78,160.02 | C33.1 19.05,160.02 | C48.+ 17.78,160.02 | 17.78,160.02 16.51,160.02 15.24,158.75 L21.1
GEHAEUSEMASSE  (via drill 0.8)
  Top 0.813: X6.GND@2 7.19,89.33 v7.62,88.9 | v7.62,81.28 7.19,80.85 X6.GND@4 | v3.81,17.78 3.56,18.03 X2.GND@4 | X2.GND@2 3.81,28.63 v3.81,30.48 | X1.GND@4 3.81,36.14 v3.81,34.29 | X1.GND@2 3.99,44.45 v7.62,44.45 | X7.GND@4 2.54,63.32 v2.54,62.23 | X7.GND@2 3.81,73.08 v3.81,74.93 | GEHAEUSE1.P$2 R58.1
  Bottom 0.813: v7.62,88.9 7.19,89.33 X6.GND@2 X6.GND@4 | X6.GND@4 7.19,80.85 v7.62,81.28 | X6.GND@4 X7.GND@2 | X7.GND@2 X7.GND@4 | X7.GND@4 5.08,62.81 5.08,53.34 6.35,52.07 6.35,46.41 X1.GND@2 | X1.GND@2 X1.GND@4 | X1.GND@4 X2.GND@2 | X2.GND@2 X2.GND@4 3.81,19.63 v3.81,17.78 5.08,16.51 5.08,5.08 6.35,3.81 16.51,3.81 17.78,5.08 GEHAEUSE1.P$2 | v3.81,30.48 3.56,30.23 X2.GND@2 | v3.81,34.29 3.56,34.54 X1.GND@4 | v7.62,44.45 7.19,44.88 X1.GND@2 | v2.54,62.23 3.56,63.25 X7.GND@4 | v3.81,74.93 3.56,74.68 X7.GND@2
GND  (via drill 0.6, 0.8)
  Top 0.406: C42.1 v181.61,172.72 | C41.2 v186.69,172.72 | C43.1 v181.61,135.89 | C44.2 v186.69,135.89 | C62.1 v181.61,97.79 | C63.2 v186.69,97.79 | T2.3 v127,88.9 C8.1 | R47.1 v24.13,29.84 | R24.2 v63.5,27.94 | R31.2 v83.82,11.43 | C51.2 v73.66,12.7 | R36.1 v22.86,166.37 | v19.05,144.78 19.01,144.74 JP1.P$4 13.93,144.74 12.7,143.51 12.7,140.97 13.97,139.7 13.93,139.7 JP1.P$2 | SJ12.2 v86.36,152.4 | R44.1 v62.23,146.05 | R45.1 v66.04,148.59 | T1.3 135.89,167.64 v135.89,165.1 | R4.1 v140.97,171.45 | R10.1 154.74,110.69 v154.94,110.49 | X1.SIGNAL v7.62,40.64 | R51.1 v41.91,173.99 | C1.2 v85.09,123.19 85.09,120.67 U1.5 86.63,120.38 87.63,119.38 | SJ46.2 v38.1,125.73 | SJ47.2 v38.1,121.92 | S2.2 v10.16,57.15 5.08,57.15 S2.4 | IC3.9 147.65,116.52 IC3.13 147.32,115.57 146.96,115.21 IC3.6 | IC10.4 92.08,99.69 v92.71,100.33 | 87.63,119.38 86.63,118.38 U1.8 85.09,118.09 v85.09,116.84 | U1.4 U1.3 87.95,119.7 87.63,119.38 | R32.2 v81.28,102.87 | C64.2 v85.09,92.71 | TSV2.C v10.79,20.32 | TSV3.C v10.79,23.5 | S3.3 12.7,8.89 11.43,7.62 3.81,7.62 2.54,8.89 S3.4 | R54.2 v12.7,167.64 | R53.2 v12.7,172.72 | SJ11.2 v35.56,95.25 | IC14.6 v52.7,133.35 | SJ41.1 v161.29,115.57
  Top 0.813: C55.2 v54.61,133.35 | C38.2 v49.53,133.35 | C34.1 v143.51,123.19 | C59.1 v140.97,119.38 | C49.2 v39.37,20.32 | C23.2 v49.53,27.94 | C27.2 v102.87,22.86 | C25.2 v67.31,24.13 | C57.2 90.37,9.96 v91.44,8.89 | C31.2 v22.86,157.48 | C33.2 v19.05,152.4 | C28.2 v31.75,140.97 | C35.2 v104.14,140.97 | C54.2 v104.14,151.13 | C61.1 v158.75,163.83 | R49.2 v41.91,182.88 | R12.2 36.83,186.69 | R13.2 36.83,186.69 | 36.83,186.69 v36.83,185.42 | 147.32,115.57 v147.32,113.03 | TSV1.C v25.4,76.2
  Route2 0.254: 43.18,95.25 48.26,95.25 | 54.61,83.82 54.61,90.17 | 60.96,95.25 66.04,95.25 | 54.61,107.95 54.61,101.6 | 76.2,97.79 81.28,97.79 | 87.63,91.44 87.63,86.36 | 93.98,97.79 99.06,97.79 | 87.63,104.14 87.63,114.3 | 76.2,120.65 81.28,120.65 | 87.63,127 87.63,132.08 | 93.98,120.65 99.06,120.65
  other vias: 146.69,91.44 105.41,85.09 58.42,13.97 53.34,114.3 105.41,96.52 29.21,92.71 110.49,68.58 110.49,53.34 100.33,42.55 116.84,46.99 119.38,46.99 121.92,46.99 129.54,46.99 116.84,52.07 116.84,57.15 116.84,59.69 129.54,58.42 129.54,55.88 129.54,49.53 116.84,64.77 131.44,99.69 135.25,99.69 139.06,99.69 139.7,97.79 139.7,92.08 129.54,90.17 139.7,95.89 133.99,85.72 137.16,85.72 147.32,120.02 149.22,113.67 145.41,113.67 147.32,109.86 149.22,109.86 145.41,120.02 149.22,120.02 156.21,166.37 156.21,168.91 156.21,177.8 143.51,176.53 143.51,173.99 143.51,166.37 143.51,168.91 143.51,171.45 158.75,168.91 158.75,166.37 156.21,163.83 156.21,161.29 137.16,147.32 138.43,148.59 139.7,148.59 137.16,148.59 138.43,147.32 139.7,147.32 133.35,152.4 143.51,152.4 144.78,152.4 132.08,152.4 154.31,91.44 156.21,91.44 152.4,96.52 154.31,96.52 156.21,96.52 158.12,96.52 150.5,96.52 148.59,96.52 146.69,96.52 144.78,96.52 142.88,96.52 142.88,92.71 133.35,99.69 137.16,99.69 129.54,99.69 129.54,95.89 129.54,93.98 129.54,92.08 129.54,88.27 143.51,120.02 116.84,62.23 116.84,54.61 116.84,49.53 124.46,46.99 127,46.99 129.54,60.96 129.54,63.5
  pour Route2 (isolate 0.406): 1.27,189.23 215.9,189.23 215.9,1.27 1.27,1.27
  pour Top (isolate 0.406): 1.27,189.23 215.9,189.23 215.9,1.27 1.27,1.27
  pour Bottom (isolate 0.406): 215.9,1.27 1.27,1.27 1.27,189.23 215.9,189.23
IC5_V+
  Top 0.813: L13.1 74.93,30.48 | 74.93,30.48 74.93,24.13 | 74.93,24.13 74.93,20.32 74.3,19.68 IC5.7 | C26.+ 74.93,30.48 | C25.1 74.93,24.13
IC5_V-
  Top 0.813: IC5.4 65.41,17.14 64.77,16.51 64.77,12.7 | 64.77,12.7 64.77,11.43 66.04,10.16 68.58,10.16 | 68.58,10.16 76.2,10.16 76.83,9.53 C52.- | C51.1 64.77,12.7 | L17.2 68.58,6.73 68.58,10.16
IC6_V+
  Top 0.813: IC6.7 94.61,19.68 95.25,20.32 95.25,22.86 | 95.25,22.86 95.25,24.13 93.98,25.4 92.71,25.4 | 92.71,25.4 L14.1 | C37.+ 92.71,25.4 | C27.1 95.25,22.86
IC6_V-
  Top 0.406: C57.1 88.7,12.7
  Top 0.813: IC6.4 86.36,17.14 86.36,12.7 | 86.36,12.7 86.36,6.35 | 88.7,12.7 86.36,12.7 | 86.36,6.35 C58.- | L20.2 88.9,3.81 86.36,6.35
INA2_V+
  Top 0.813: 96.52,142.24 96.52,143.51 97.16,144.15 IC16.8 | 96.52,142.24 96.52,140.97 | C35.1 96.52,140.97 | L11.1 97.79,137.16 96.52,138.43 96.52,140.97 | C53.+ 96.52,142.24
INA2_V-
  Top 0.406: L18.2 97.79,154.94
  Top 0.813: 96.52,151.13 96.52,148.59 97.16,147.96 IC16.5 | 96.52,151.13 C54.1 | C68.- 96.52,151.13 | 97.79,154.94 96.52,153.67 96.52,151.13
INA_V+
  Top 0.406: 50.16,127.43 C38.1 | 49.94,124.84 IC14.8
  Top 0.813: IC14.8 50.16,127.43 | L15.1 46.61,124.84 | 46.61,124.84 C46.+ | 46.61,124.84 49.94,124.84
INA_V-
  Top 0.406: 53.98,127.43 C55.1 | 54.2,124.84 IC14.5
  Top 0.813: IC14.5 53.98,127.43 | L19.2 57.53,124.84 | 57.53,124.84 C56.- | 57.53,124.84 54.2,124.84
LD-ANODE
  Top 0.813: X7.SIGNAL 10.16,68.58 | 10.16,68.58 12.7,68.58 | 12.7,68.58 21.59,68.58 | 21.59,67.31 L1.P$2 20.95,60.96 16.51,60.96 15.24,59.69 15.24,44.45 16.51,43.18 SJ51.1 | SJ6.1 10.16,68.58 | SJ5.2 12.7,68.58 | TSV1.A 25.4,68.58 24.13,67.31 21.59,67.31 | LASORB1.LDA 21.59,68.58 | 21.59,68.58 21.59,67.31 | SJ50.1 12.7,68.58
LT1028_V+
  Top 0.813: IC17.7 41.27,27.3 41.91,27.94 | C23.1 41.91,27.94 | L12.1 40.64,31.75 41.91,30.48 | 41.91,30.48 41.91,27.94 | C24.+ 41.91,30.48
LT1028_V-
  Top 0.406: 34.29,20.52 C49.1
  Top 0.813: L16.2 34.29,22.86 | IC17.4 34.29,22.86 | 34.29,22.86 41.27,22.86 42.55,21.59 C50.- | 34.29,22.86 34.29,20.52
MODULATION  (via drill 0.8)
  Top 0.406: SJ5.1 v12.7,63.5
  Bottom 0.406: v12.7,63.5 12.7,62.23 15.24,59.69 15.24,43.18 8.89,36.83 8.89,11.43 S3.1
N$1
  Top 0.406: 93.98,49.53 95.25,49.53 | 95.25,49.53 96.52,49.53 | 96.52,49.53 C13.1 | 93.98,49.53 92.71,49.53 91.44,50.8 91.44,60.96 90.17,62.23 X3.6 | TP8.TP 93.98,49.53 | 95.25,49.53 95.56,49.84 95.56,52.7 R59.2 | C6.- 99.69,52.7 96.52,49.53
N$2
  Top 0.406: T1.1 132.25,171.45 | 132.25,171.45 129.54,171.45 128.27,170.18 D2.ANODE | 132.25,171.45 135.89,171.45 | 135.89,171.45 137.16,171.45 138.43,170.18 R3.2 | C19.2 135.89,171.45
N$3
  Top 0.406: T1.2 132.25,164.93 133.35,163.83 | 133.35,163.83 138.43,163.83 | 138.43,163.83 140.97,163.83 | 140.97,163.83 142.24,163.83 | R3.1 138.43,163.83 | R1.1 142.24,163.83 | D16.ANODE 138.43,163.83 | 142.24,163.83 146.05,163.83 147.32,162.56 IC1.1 | 133.35,163.83 133.35,161.29 132.72,160.66 C2.+ | R4.2 140.97,163.83
N$4
  Top 0.406: IC2.1 57.15,110.49 55.88,111.76 55.88,113.03 SJ48.1
N$5
  Top 0.406: D2.KATHODE 128.27,154.94 129.54,153.67 138.43,153.67 | 138.43,153.67 142.24,153.67 | 142.24,153.67 149.86,153.67 | D16.KATHODE 138.43,153.67 | R1.2 142.24,153.67
  Top 0.813: R2.2 146.05,151.13 | C4.+ 146.05,151.13 | 148.59,151.13 149.86,152.4 149.86,153.67 IC1.2 | 148.59,151.13 146.05,151.13 | D1.ANODE 148.59,151.13
N$6
  Top 0.406: SJ35.1 62.23,137.16 | 62.23,137.16 65.84,137.16 R37.1 | R44.2 62.23,137.16
N$7
  Top 0.406: IC2.2 54.61,100.33 | SJ23.1 34.29,101.6 34.29,104.14 | 34.29,104.14 34.29,106.68 | 34.29,106.68 SJ21.1 | R46.1 34.29,104.14 | R5.2 49.53,100.33 54.61,100.33 | 54.61,100.33 54.61,107.95 35.56,107.95 34.29,106.68
N$8
  Top 0.406: C7.- 97.79,66.67 | L23.1 95.5,64.14 95.25,64.14 95.25,66.67 | C12.1 99.06,60.96 97.79,62.23 97.79,66.67 | 97.79,66.67 95.25,66.67 | 95.25,66.67 R62.2
N$9
  Top 0.406: R10.2 R68.1
N$10
  Top 0.406: R8.1 78.74,163.83 80.01,162.56 R38.1
N$11
  Top 0.406: R34.1 R37.2
N$12
  Top 0.406: R38.3 85.09,162.56 86.36,163.83 R9.2
N$13
  Top 0.406: SJ62.2 R14.2
N$14
  Top 0.406: 86.36,146.69 83.82,146.69 82.55,147.96 SJ20.1 | SJ12.1 86.36,146.69 | IC16.6 86.36,146.69
N$15
  Top 0.406: R43.1 R34.2
N$16
  Top 0.813: SJ29.2 197.61,160.15 L2.P$2 193.04,153.03 C15.+ 193.04,136.96 C44.1 | C44.1 191.77,135.69 L6.P$1 | C44.1 SJ30.1
N$17
  Top 0.813: R12.1 27.94,186.69 26.67,187.96 13.97,187.96 12.7,186.69 12.7,181.61 13.84,180.47 S1.4
N$18
  Top 0.813: S1.1 15.24,185.42 16.51,186.69 25.4,186.69 27.94,184.15 40.64,184.15 42.11,185.62 R13.1
N$19
  Top 0.406: SJ20.2 R38.2
N$20
  Top 0.406: IC17.2 36.2,27.3 37.47,26.04 IC17.6 41.27,26.04 41.91,25.4 49.53,25.4 | 49.53,25.4 SJ32.1 | TP9.TP 49.53,22.86 49.53,25.4
N$21
  Top 0.406: R55.2 24.13,26.67 | 24.13,26.67 R33.1 | 24.13,26.67 20.95,23.5 TSV3.A
N$22
  Top 0.406: SJ27.1 74.93,137.16 76.2,138.43 76.2,145.41 | 76.2,145.41 76.2,149.86 | 76.2,149.86 76.2,156.21 74.93,157.48 SJ34.1 | SJ33.1 76.2,149.86 | IC16.7 76.2,145.41
N$23
  Top 0.406: SJ17.2 15.24,17.78 | 15.24,17.78 SJ49.1 | TSV2.A 15.24,20.14 15.24,17.78
N$24
  Top 0.813: R19.1 151.13,93.98 | 151.13,93.98 R18.2 | C5.+ 151.13,93.98
N$25
  Top 0.813: D5.KATHODE 123.19,97.79 | 123.19,97.79 SJ4.1 | C8.2 127,97.79 | 127,97.79 123.19,97.79 | Q2.3 134.86,96.28 133.35,97.79 127,97.79
N$26
  Top 0.813: R18.1 Q2.2 Q2.4
N$27
  Top 0.406: R22.1 144.78,87.43 | 144.78,87.43 142.24,87.43 | C9.+ 142.24,87.43 | 142.24,87.43 133.15,87.43 | 133.15,87.43 132.08,86.36 132.08,85.09 130.81,83.82 128.12,83.82 T2.2 | 133.15,87.43 R21.2 | R20.1 144.78,87.43
N$28
  Top 0.406: R21.1 137.12,89.93 Q2.1
N$29
  Top 0.406: C10.2 122.99,83.82 R23.2 125.68,83.62
  Top 0.813: 125.68,83.62 T2.1
N$30
  Top 0.813: SJ2.2 158.75,93.98 | 158.75,93.98 R19.2 | R22.2 158.75,93.98
N$31
  Top 0.406: R23.1 D5.ANODE
N$32
  Top 0.406: R39.1 140.97,58.42 | 140.97,58.42 138.43,58.42 135.89,60.96 134.62,60.96 | C40.+ 134.62,60.96 | 140.97,58.42 R40.2 R40.1 | 134.62,60.96 132.08,60.96 | 132.08,60.96 130.81,62.23 130.81,64.77 Q3.1 | 132.08,60.96 D3.3
N$33
  Top 0.813: R2.1 132.08,151.13 | 132.08,151.13 SJ3.1 | C18.+ 132.08,151.13
N$34
  Top 0.406: R25.2 76,13.97 74.93,13.97 73.66,15.24 71.12,15.24 69.85,16.51 69.85,19.05 69.22,19.68 IC5.2 64.14,19.68 63.5,20.32 R24.1 63.5,22.86
N$35
  Top 0.406: 80.01,18.41 80.64,18.41 81.28,19.05 81.28,20.12 R30.2 | 80.01,18.41 76.2,18.41 | 76.2,18.41 IC5.6 | 80.01,18.41 R26.1 | R25.1 76.2,18.41
N$36
  Top 0.406: IC6.6 96.95,18.41 | 96.95,18.41 R28.2 | 96.95,18.41 96.95,17.35 97.79,16.51 97.79,14.17 R29.1 97.99,9.96 C11.2
N$37
  Top 0.406: SJ26.1 40.64,116.84 | 40.64,116.84 SJ25.2 | SJ24.2 40.64,111.76 40.64,116.84
N$38
  Top 0.406: IC6.3 84.45,18.41 83.82,17.78 R31.1
N$39
  Top 0.406: R30.1 84.66,19.68 IC6.2 89.53,19.68 90.17,19.05 90.17,16.51 92.71,13.97 | 92.71,13.97 R29.2 | C11.1 92.71,10.16 92.71,13.97
N$40
  Top 0.813: S1.2 19.05,184.15 21.59,181.61 27.48,181.61 T4.3
N$41
  Top 0.406: R14.1 30.48,15.24 | 30.48,15.24 11.43,15.24 10.16,13.97 S3.2 | SJ60.2 31.75,10.16 30.48,11.43 30.48,15.24
N$42  (via drill 0.8)
  Top 0.406: R26.2 v80.01,10.16 | IC5.3 64.14,18.41 63.5,17.78 v63.5,10.16 SJ60.1 | v101.6,10.16 102.87,11.43 R27.1
  Bottom 0.406: v63.5,10.16 v80.01,10.16 v101.6,10.16
N$43
  Top 0.406: SJ49.2 43.18,17.78 | 43.18,17.78 55.88,17.78 | 55.88,17.78 55.88,24.13 54.61,25.4 SJ32.2 | 55.88,17.78 SJ16.1 | SJ62.1 41.91,15.24 43.18,16.51 43.18,17.78
N$44
  Top 0.406: S2.3 12.7,57.15 10.16,59.69 SJ6.2
N$45
  Top 0.406: 151.13,117.81 | IC3.10 151.13,117.17 | 151.13,117.17 | IC3.11 151.13,117.81 | 151.13,117.81 151.13,118.11 151.13,118.47 IC3.12
  Top 0.813: 151.13,117.17 151.13,118.11 151.13,121.28 | 151.13,121.28 151.13,123.19 | 151.13,123.19 151.13,132.04 | 151.13,132.04 C69.2 | C34.2 151.13,123.19 | SJ7.1 137.16,109.22 138.43,110.49 138.43,119.38 140.34,121.28 151.13,121.28 | 151.13,132.04 151.13,135.89 149.86,137.16 SJ8.1
N$46
  Top 0.813: SJ8.2 138.43,137.16 | 138.43,137.16 133.35,137.16 132.08,135.89 L22.P$1 | C73.+ 139.7,130.81 138.43,132.08 138.43,137.16
N$47
  Top 0.406: U1.6 83.5,119.7 82.55,120.65 82.55,124.46 83.82,125.73 101.6,125.73 C66.+
N$48
  Top 0.406: R7.3 R7.1 26.67,111.76 R56.2
N$49
  Top 0.813: SJ51.2 20.32,43.18 21.59,44.45 L1.P$1 21.59,54.61 22.86,55.88 29.21,55.88 | X4.8 30.48,54.61 29.21,55.88 | X4.7 30.48,57.15 29.21,55.88
N$50
  Top 0.813: SJ7.2 120.65,109.22 119.38,110.49 119.38,111.76 | SJ9.2 120.65,113.03 119.38,111.76 | SJ57.1 119.38,111.76
N$51
  Top 0.406: C3.- 160.02,121.92 161.29,120.65 SJ41.2
N$52
  Top 0.406: IC17.3 31.32,26.04 R33.2
N$53
  Top 0.406: SJ27.2 68.38,137.16 R41.2
N$54
  Top 0.406: LED3.A R54.1
N$55
  Top 0.813: L21.2 15.24,149.86 | 15.24,149.86 JP1.P$5 | C28.1 24.13,140.97 22.86,142.24 22.86,147.32 | 22.86,147.32 22.86,148.59 21.59,149.86 15.24,149.86 | C36.+ 22.86,147.32 | TP11.TP 22.86,147.32
N$56
  Top 0.406: 29.21,162.56 R35.1 30.48,162.56 | R36.2 29.21,166.37 30.48,165.1 30.48,162.56 | 30.48,162.56 IC4.1
N$57
  Top 0.406: R11.2 88.27,102.87 | 88.27,102.87 R32.1 | IC10.5 87,99.69 88.27,100.97 88.27,102.87
N$58
  Top 0.406: SJ38.2 55.09,119.38 IC14.4
N$59
  Top 0.813: 134.62,67.31 L5.P$2 | C39.+ 134.62,67.31 | 134.62,67.31 132.08,67.31 130.81,68.58 130.81,71.12 129.54,72.39 124.46,72.39 123.19,71.12 Q3.2
N$60
  Top 0.406: R39.2 153.67,58.42 154.94,59.69 154.94,67.31
  Top 0.813: L5.P$1 154.94,67.31 SJ14.2
N$61
  Top 0.406: D3.1 130.64,52.24 120.65,62.23 Q3.3
  Top 0.813: SJ15.1 Q3.3
N$62
  Top 0.406: SJ33.2 70.92,149.86 R42.2
N$63
  Top 0.406: R42.1 69.85,154.94 68.58,156.21 66.04,156.21 | SJ40.1 62.23,151.13 63.5,152.4 63.5,154.94 64.77,156.21 66.04,156.21 | R45.2 66.04,156.21
N$64  (via drill 0.8)
  Top 0.406: SJ23.2 v24.13,101.6
  Bottom 0.406: R6.1 17.78,102.87 19.05,101.6 v24.13,101.6
N$65  (via drill 0.8)
  Top 0.406: R27.2 v102.87,19.05 R28.1 | SJ16.2 v62.23,17.78
  Bottom 0.406: v102.87,19.05 101.6,17.78 v62.23,17.78
N$66
  Top 0.406: SJ21.2 R16.1
N$67  (via drill 0.8)
  other vias: 38.1,114.3
N$69
  Top 0.406: R41.1 R43.2
N$70
  cutout Top: 196.85,1.27 196.85,11.43 215.9,11.43 215.9,1.27
N$71  (via drill 0.8)
  Top 0.406: SJ39.1 v25.4,97.79 | v51.44,128.27 IC14.7
  Bottom 0.406: v51.44,128.27 51.44,109.86 50.8,109.22 26.67,109.22 25.4,107.95 v25.4,97.79
N$72  (via drill 0.8)
  Top 0.406: SJ44.1 38.1,128.27 v39.37,129.54 39.37,130.81 | R66.1 39.37,130.81 | SJ19.2 67.31,121.92 | 67.31,121.92 67.31,99.06 68.58,97.79 SJ37.2 | 67.31,121.92 v67.31,128.27 | 39.37,130.81 39.37,132.08 38.1,133.35 SJ45.1
  Bottom 0.406: v67.31,128.27 66.04,129.54 v39.37,129.54
N$73
  Bottom 0.813: ST1.A18 ST1.C18 201.93,135.89 198.12,139.7 198.12,181.61 195.58,184.15 27.94,184.15 22.86,179.07 S1.6
N$74
  Top 0.406: R15.1 30.48,111.76 30.48,110.49 29.21,109.22 R17.2
N$77
  Top 0.406: SJ24.1 34.29,111.76 34.29,111.96 R15.2
N$79
  Top 0.406: SJ25.1 R7.2
N$80
  cutout Route2: 196.85,11.43 196.85,1.27 215.9,1.27 215.9,11.43
N$81
  Top 0.813: L8.2 43.18,151.13 | 43.18,151.13 43.18,147.32 44.45,146.05 C30.+ | L4.1 43.18,151.13
N$82
  cutout Bottom: 215.9,11.43 215.9,1.27 196.85,1.27 196.85,11.43
N$83
  Top 0.406: R56.1 22.86,111.76 R6.2
N$84
  Top 0.406: SJ11.1 40.64,95.25 40.64,97.79 | SJ10.1 40.64,97.79 | 40.64,97.79 49.53,97.79 R5.1
N$85
  Top 0.406: 21.59,109.22 R17.1 20.32,109.22 | R6.3 20.32,109.22 | 20.32,109.22 20.32,106.68 | 20.32,106.68 20.32,104.14 | 20.32,104.14 20.32,102.87 22.86,100.33 SJ22.1 | R46.2 20.32,104.14 | R16.2 20.32,106.68
N$86
  Top 0.406: 46.99,174.19 46.99,175.26 45.72,176.53 41.91,176.53 40.64,175.26 38.25,175.26 T3.1 | R51.2 R52.1
  Top 0.813: 46.99,174.19 R51.2
N$87
  cutout Route3: 196.85,1.27 196.85,11.43 215.9,11.43 215.9,1.27
N$88
  Top 0.406: L24.2 R62.1
N$89  (via drill 0.8)
  Top 0.406: 46.99,182.68 v46.99,180.34 | v34.92,179.71 31.27,179.71 T4.1
  Top 0.813: R50.2 R49.1 46.99,182.68
  Bottom 0.406: v46.99,180.34 35.56,180.34 v34.92,179.71
N$90
  Top 0.406: R59.1 L23.2
N$93
  cutout Bottom: 77.47,107.95 77.47,87.63 97.79,87.63 97.79,107.95
N$94
  cutout Bottom: 77.47,130.81 77.47,110.49 97.79,110.49 97.79,130.81
N$96
  cutout Route3: 44.45,106.68 64.77,106.68 64.77,85.09 44.45,85.09
N$97
  Top 0.813: S1.5 21.72,176.53 T3.3
N$98
  cutout Route3: 77.47,107.95 77.47,87.63 97.79,87.63 97.79,107.95
N$99
  cutout Route2: 44.45,106.68 44.45,85.09 46.99,85.09 46.99,106.68
N$100
  cutout Route2: 44.45,88.9 64.77,88.9 64.77,85.09 44.45,85.09
N$101
  cutout Route2: 64.77,85.09 64.77,106.68 62.23,106.68 62.23,85.09
N$102
  cutout Route2: 64.77,102.87 44.45,102.87 44.45,106.68 64.77,106.68
N$103
  Top 0.406: SJ13.2 14.61,26.67 | 14.61,26.67 R55.1 | R47.2 15.24,29.84 14.61,29.21 14.61,26.67
N$104
  Top 0.406: IC10.6 83.19,98.42 82.55,97.79 | 82.55,97.79 SJ37.1 | R57.2 83.82,85.09 82.55,86.36 82.55,97.79
N$105
  cutout Route3: 77.47,130.81 77.47,110.49 97.79,110.49 97.79,130.81
N$106
  Top 0.406: 93.98,99.06 93.98,101.8 R11.1 | 93.98,99.06 93.98,97.79 | R57.1 92.71,85.09 93.98,86.36 93.98,92.71 | 93.98,92.71 93.98,97.79 | SJ36.1 93.98,99.06 | IC10.2 93.34,97.16 93.98,97.79 | C64.1 93.98,92.71
N$107
  cutout Top: 44.45,106.68 44.45,85.09 64.77,85.09 64.77,106.68
N$108  (via drill 0.8)
  Top 0.813: X6.SIGNAL v8.89,85.09 | v107.95,78.74 v111.76,78.74 | v199.39,129.54 R67.1
  Bottom 0.813: X5.3 12.7,111.76 15.24,109.22 15.24,85.09 | 15.24,85.09 v8.89,85.09 | 15.24,85.09 19.05,81.28 26.67,81.28 27.94,82.55 40.64,82.55 41.91,81.28 105.41,81.28 v107.95,78.74 | v111.76,78.74 114.3,76.2 180.34,76.2 200.66,96.52 200.66,128.27 v199.39,129.54
N$109
  Top 0.813: SJ42.1 53.34,91.44 IC2.3
N$111
  Top 0.406: SJ13.1 8.89,26.67 7.62,25.4 7.62,24.13 | 7.62,24.13 7.62,19.05 8.89,17.78 SJ17.1 | X2.SIGNAL 7.62,24.13
N$112
  cutout Top: 77.47,107.95 77.47,87.63 97.79,87.63 97.79,107.95
N$117
  Top 0.813: SJ43.2 53.34,88.9 IC2.4
N$118
  Top 0.406: SJ18.1 92.71,119.38 | 92.39,119.06 91.71,118.38 U1.1 | 92.39,119.06 92.71,119.38 | C1.1 91.44,123.19 92.71,121.92 92.71,119.38 | 92.39,119.06 U1.2
N$119
  Top 0.406: U1.7 83.5,119.06 82.55,118.11 81.28,118.11 | 81.28,118.11 71.16,118.11 C65.1 | SJ19.1 80.01,121.92 81.28,120.65 81.28,118.11
N$120
  cutout Route2: 77.47,107.95 77.47,87.63 80.01,87.63 80.01,107.95
N$121
  Top 0.406: R61.3 R61.1 R60.2
N$122
  cutout Route2: 77.47,90.17 77.47,87.63 97.79,87.63 97.79,90.17
N$123
  cutout Route2: 95.25,87.63 95.25,107.95 97.79,107.95 97.79,87.63
N$124
  cutout Route2: 97.79,105.41 77.47,105.41 77.47,107.95 97.79,107.95
N$125
  Top 0.406: SJ45.2 19.05,133.35 17.78,132.08 R60.1
N$126
  Top 0.406: R64.1 SJ44.2
N$127
  Top 0.406: R65.2 R63.1
N$128
  Top 0.406: R63.2 SJ46.1
N$129
  Top 0.406: R61.2 SJ47.1
N$130
  Top 0.813: SJ50.2 12.7,90.17 5.08,97.79 5.08,107.99 X5.8
N$131
  cutout Top: 77.47,110.49 77.47,130.81 97.79,130.81 97.79,110.49
N$135
  Top 0.406: C31.1 29.21,157.48 | D17.KATHODE 33.02,153.67
  Top 0.813: 33.02,157.48 C31.1 | 33.02,157.48 33.02,153.67 33.02,151.13 | 33.02,151.13 33.02,147.32 34.29,146.05 C32.+ | L4.2 33.02,151.13 | IC4.3 33.02,157.48
N$138
  Top 0.406: C70.2 152.4,115.57 | R68.2 152.4,115.57 | C3.+ 153.03,118.75 152.4,118.11 152.4,115.86 | IC3.8 152.4,115.86 | 152.4,115.86 152.4,115.57
N$139
  Top 0.406: 151.13,114.3 150.22,115.22 150.21,115.21 IC3.7 | 143.87,118.47 143.51,118.11 | 143.81,117.81 143.51,118.11 | 143.84,117.17 143.51,116.84 | 143.84,116.52 143.51,116.84 | IC3.1 143.51,118.47 143.51,118.11 | IC3.2 143.51,117.81 143.51,118.11 | IC3.3 143.51,117.17 143.51,116.84 | IC3.4 143.51,116.52 143.51,116.84
  Top 0.813: 143.51,118.11 143.51,116.84 143.51,114.3 | 143.51,114.3 143.51,113.03 144.15,112.39 | 144.15,112.39 144.78,111.76 151.13,111.76 | 151.13,111.76 151.13,114.3 | C59.2 143.31,114.1 143.51,114.3 | SJ56.2 152.4,106.68 151.13,107.95 151.13,111.76 | C72.+ 142.24,110.49 144.15,112.39
N$142
  Top 0.813: SJ9.1 130.81,113.03 | 130.81,113.03 132.08,114.3 L22.P$2 | C60.+ 130.81,113.03
N$143
  cutout Bottom: 44.45,106.68 64.77,106.68 64.77,85.09 44.45,85.09
N$151
  cutout Route2: 77.47,130.81 77.47,110.49 80.01,110.49 80.01,130.81
N$152
  cutout Route2: 77.47,130.81 77.47,128.27 97.79,128.27 97.79,130.81
N$153
  cutout Route2: 95.25,130.81 95.25,110.49 97.79,110.49 97.79,130.81
N$154
  cutout Route2: 97.79,113.03 77.47,113.03 77.47,110.49 97.79,110.49
N$162
  Bottom 0.813: ST1.A14 ST1.C14 200.66,149.86 200.66,182.88 196.85,186.69 25.4,186.69 22.86,184.15 22.73,184.15 S1.3
N$173
  Top 0.813: R48.1 5.08,49.53 LED1.K
N$174
  Top 0.813: R48.2 10.49,51.74 S2.1
N$175
  Top 0.406: LED2.K R53.1
N$1111
  Top 0.406: 20.32,125.73 R60.3 22.86,119.38 50.01,119.38 IC14.1 | 20.32,125.73 20.32,128.27 | 20.32,128.27 20.32,129.54 21.59,130.81 R66.2 | R64.2 20.32,128.27 | R65.1 20.32,125.73
V+
  Top 0.813: D1.KATHODE 157.1,156.21 | IC1.3 157.1,156.21 | 157.1,156.21 158.75,156.21 | 158.75,156.21 SJ1.2 | 158.75,156.21 C61.2
V+_UNGEFILTERT  (via drill 0.8)
  Top 0.406: LED2.A 1.91,174.62 2.54,175.26 34.29,175.26 v35.56,173.99 | v40.01,176.53 40.01,177.8 | R52.2 55.88,173.99
  Top 0.813: C41.1 193.04,173.79 C14.+ v191.77,181.61 | C41.1 191.77,172.52 L2.P$1 189.87,167.64 TP1.TP | C41.1 SJ29.1 | T3.2 37.78,177.48 38.1,177.8 40.01,177.8 55.88,177.8 | L8.1 54.61,151.13 55.88,152.4 55.88,173.99 55.88,177.8 | 55.88,177.8 v57.15,179.07 | 53.34,174.19 R52.2 53.34,173.99 53.34,174.19
  Bottom 0.406: v35.56,173.99 38.1,176.53 v40.01,176.53
  Bottom 0.813: v57.15,179.07 182.88,179.07 185.42,181.61 v191.77,181.61
V-
  Top 0.813: SJ28.2 170.69,160.15 L3.P$2 175.26,153.03 C17.- 175.26,136.96 C43.2 | SJ31.1 C43.2 | C43.2 176.53,135.69 L7.P$1
V-_UNGEFILTERT  (via drill 0.8)
  Top 0.813: 175.26,176.53 C16.- v173.99,181.61 | 175.26,176.53 175.26,173.79 C42.2 | C42.2 176.53,172.52 L3.P$1 | SJ28.1 C42.2 | TP2.TP 175.26,176.53 | v57.15,181.61 55.88,182.88 R50.1 53.34,182.68 53.34,180.34 52.07,179.07 40.64,179.07 38.73,181.61 v33.02,181.61 31.26,181.61 T4.2
  Bottom 0.406: LED3.K 1.91,165.74 3.81,163.83 30.48,163.83 33.02,166.37 v33.02,181.61
  Bottom 0.813: v57.15,181.61 v173.99,181.61
V_GEREGELT
  Top 0.406: SJ18.2 106.68,119.38 107.95,118.11 107.95,99.06 | 107.95,99.06 SJ36.2 | SJ48.2 59.69,113.03 | 59.69,113.03 59.69,116.84 | 59.69,116.84 SJ26.2 | SJ38.1 59.69,119.38 59.69,116.84 | 107.95,99.06 107.95,83.82 | 59.69,113.03 59.69,99.06 64.77,93.98 73.66,93.98 74.93,92.71 74.93,86.36 78.74,82.55 106.68,82.55
  Top 0.813: C71.+ 105.41,78.11 | 105.41,78.11 105.41,72.39 | 105.41,66.67 105.41,60.96 | 105.41,60.96 105.41,55.24 | 105.41,55.24 105.41,49.53 | 105.41,49.53 C13.2 | C12.2 105.41,60.96 | C7.+ 105.41,66.67 | C6.+ 105.41,55.24 | 114.3,69.85 114.3,92.71 | 114.3,92.71 114.3,97.79 | 114.3,97.79 SJ4.2 | SJ57.2 114.3,111.76 | 114.3,111.76 114.3,97.79 | 114.3,111.76 114.3,149.86 115.57,151.13 SJ3.2 | SJ15.2 114.3,69.85 | 105.41,49.53 105.41,46.99 | 105.41,46.99 105.41,45.72 104.14,44.45 91.44,44.45 88.9,46.99 88.9,54.61 | TP5.TP 114.3,92.71 | TP7.TP 105.41,46.99 | 114.3,69.85 114.3,41.91 113.03,40.64 80.01,40.64 77.47,43.18 77.47,46.99 80.01,49.53 82.55,49.53 83.82,50.8 83.82,54.61 | C74.2 105.41,72.39 | 105.41,72.39 105.41,66.67 | 107.95,83.82 106.68,82.55 105.41,81.28 105.41,78.11 | 83.82,54.61 83.82,55.88 85.09,57.15 X3.4 87.63,57.15 88.9,55.88 88.9,54.61 | 83.82,54.61 X3.3 88.9,54.61
V_SENSE+  (via drill 0.8)
  Top 0.406: IC16.4 v108.58,147.96
  Bottom 0.406: v108.58,147.96 110.49,146.05 110.49,73.66 109.22,72.39 39.37,72.39 38.1,71.12 38.1,63.5 36.83,62.23 X4.5
V_SENSE-  (via drill 0.8)
  Top 0.406: v107.31,144.15 IC16.1
  Bottom 0.406: v107.31,144.15 109.22,142.24 109.22,76.2 107.95,74.93 38.1,74.93 36.83,73.66 36.83,68.58 35.56,67.31 X4.3
V_SOLL
  Top 0.406: 97.79,78.11 C71.- | SJ22.2 22.86,91.44 | SJ39.2 25.4,91.44 | 25.4,91.44 22.86,91.44 | 25.4,91.44 25.4,85.09 26.67,83.82 68.58,83.82 72.39,80.01 94.87,80.01 L24.1 95.63,80.01 97.79,80.01 97.79,78.11 | 22.86,91.44 20.32,91.44 19.05,92.71 TP6.TP | C74.1 99.06,72.39 97.79,73.66 97.79,78.11
(copper drawn outside any net)
  shapes: Top area x1

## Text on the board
Top: 1
Route2: 2
Route3: 3
Bottom: 4
tStop: Leibniz Universität Hannover | Institut für Quantenoptik | Jan Rasmus Holst, Steffen Sauer | Rauscharmer Lasertreiber | 2021-01-18 | Version 1 | Serie 1
Document: Display | Sollspannung | Filterung | Regelkreis/Ausgang | Spannungsregelung | Modulation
